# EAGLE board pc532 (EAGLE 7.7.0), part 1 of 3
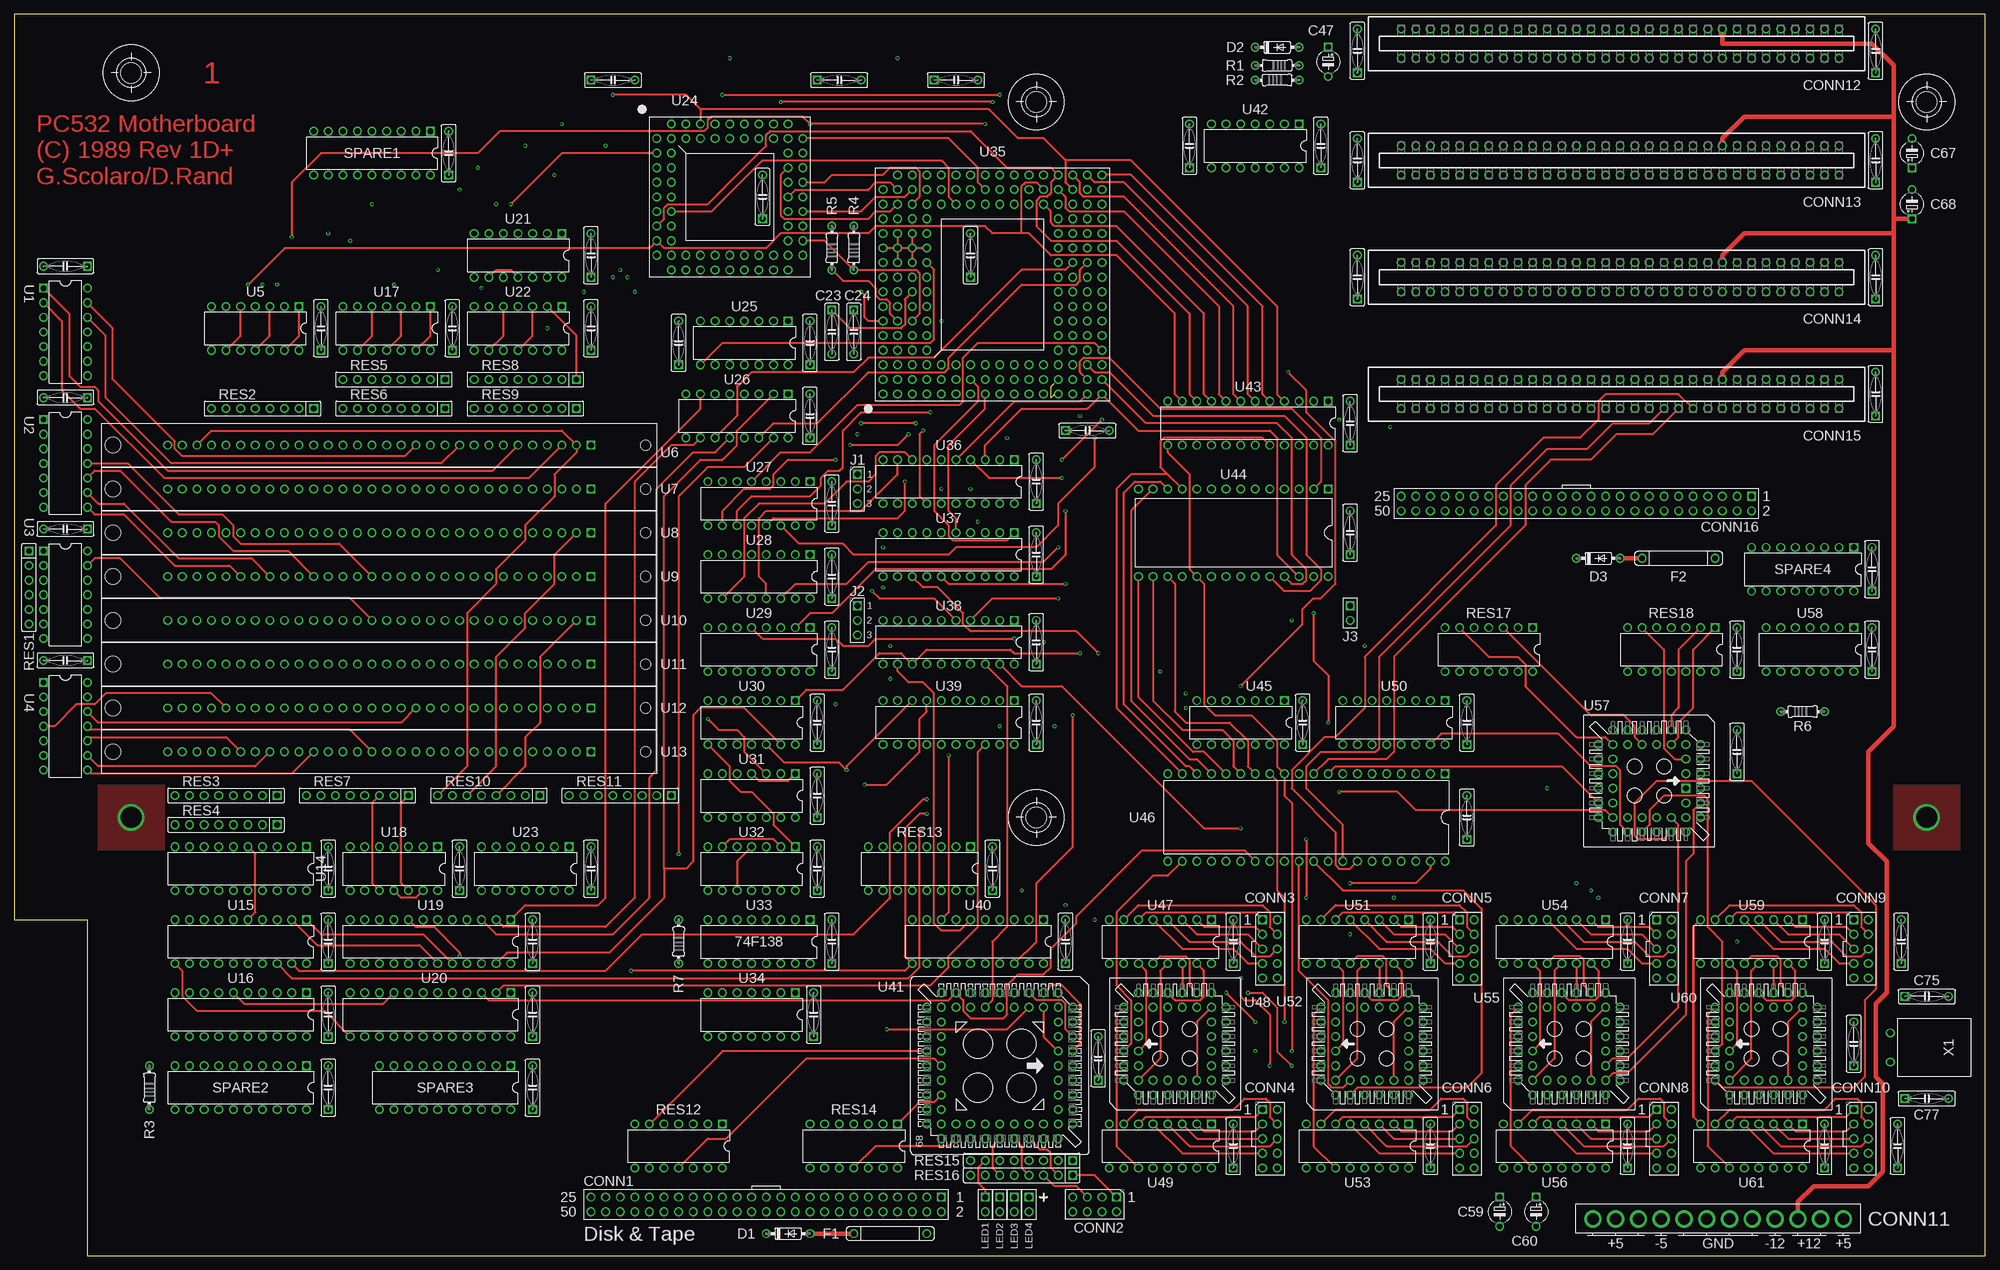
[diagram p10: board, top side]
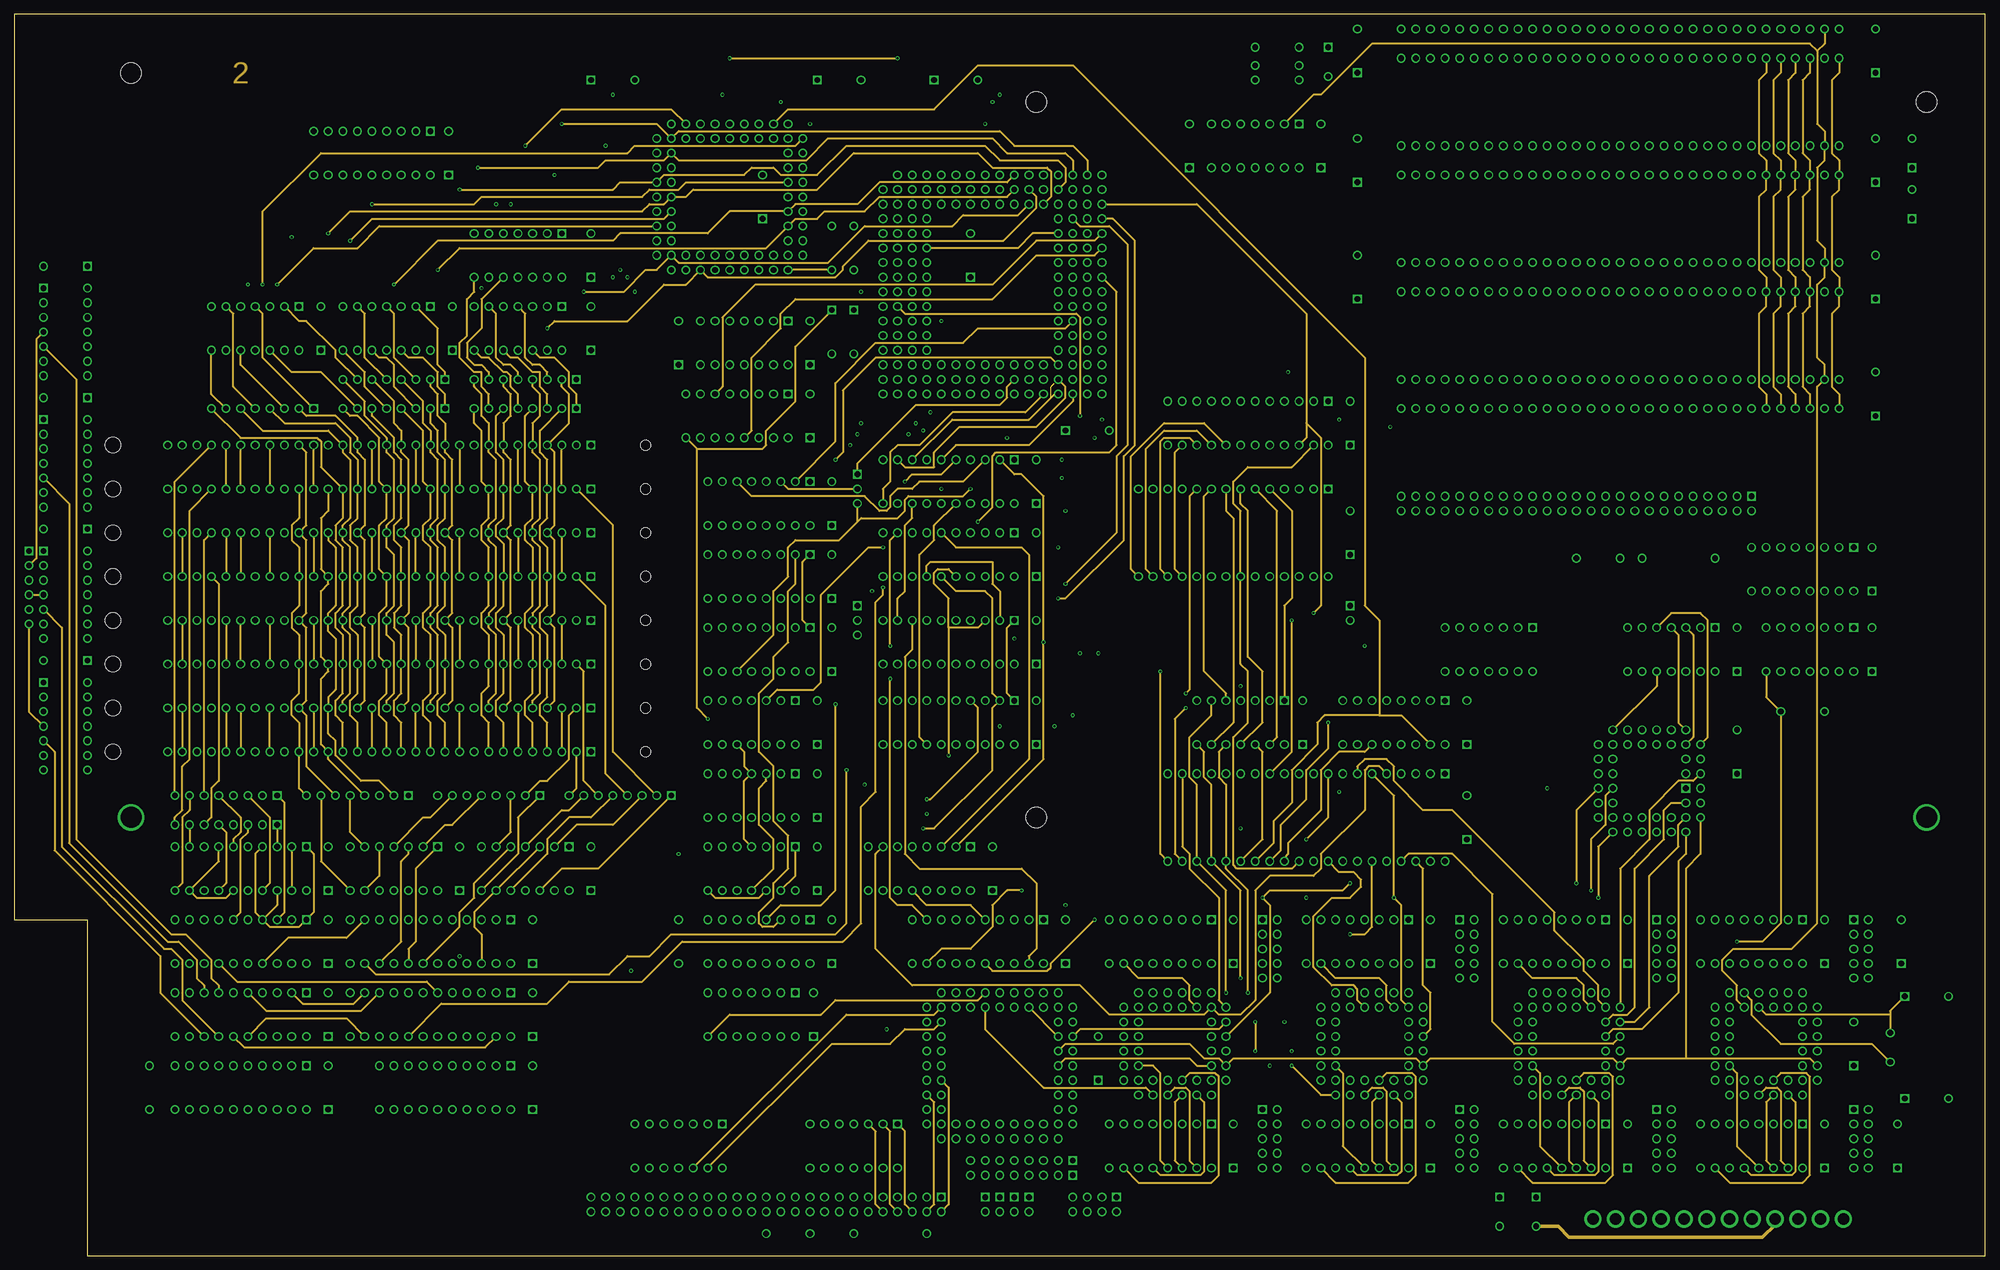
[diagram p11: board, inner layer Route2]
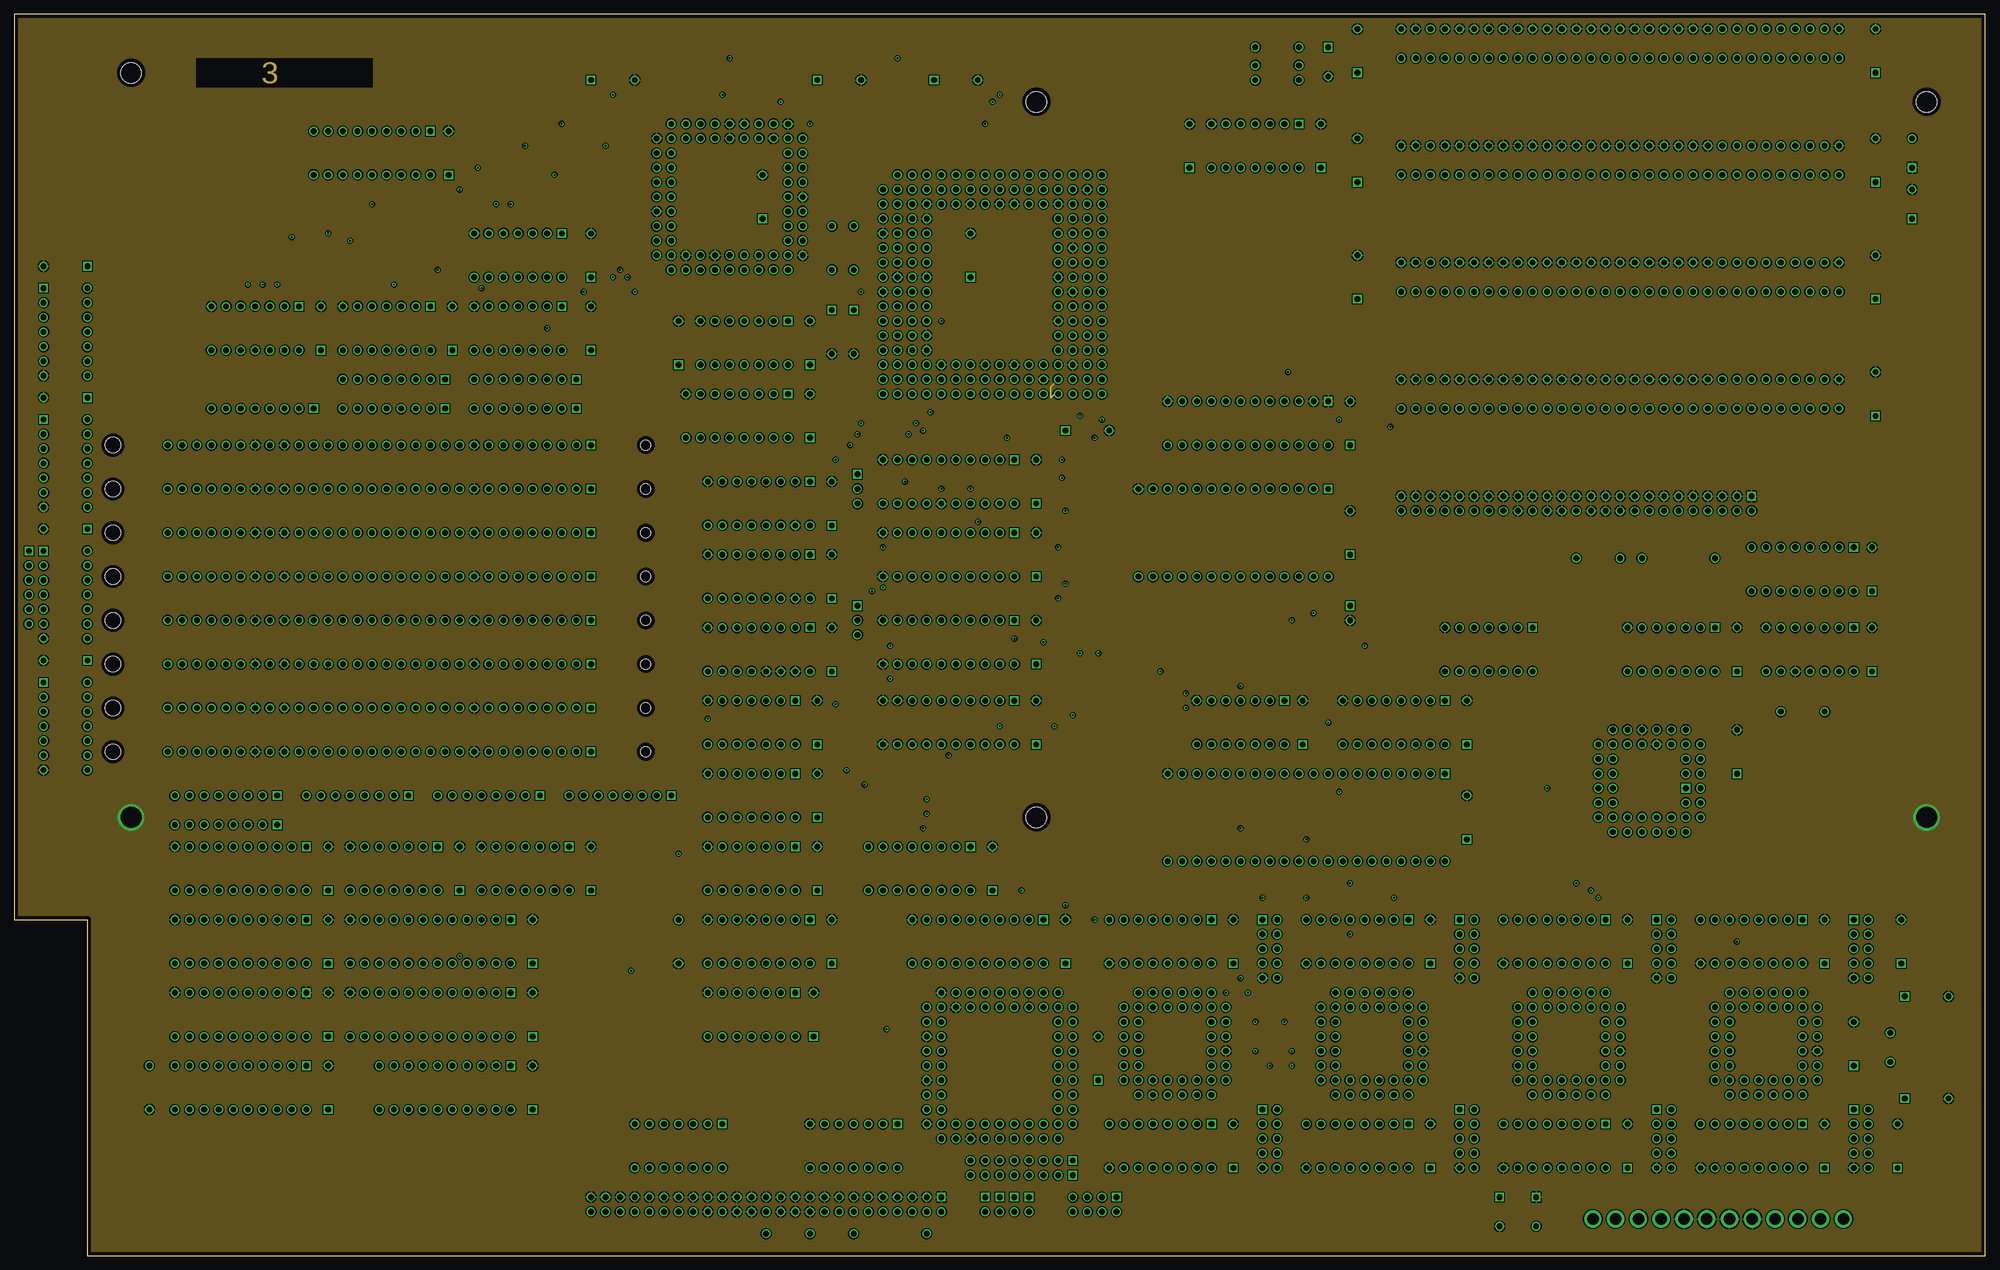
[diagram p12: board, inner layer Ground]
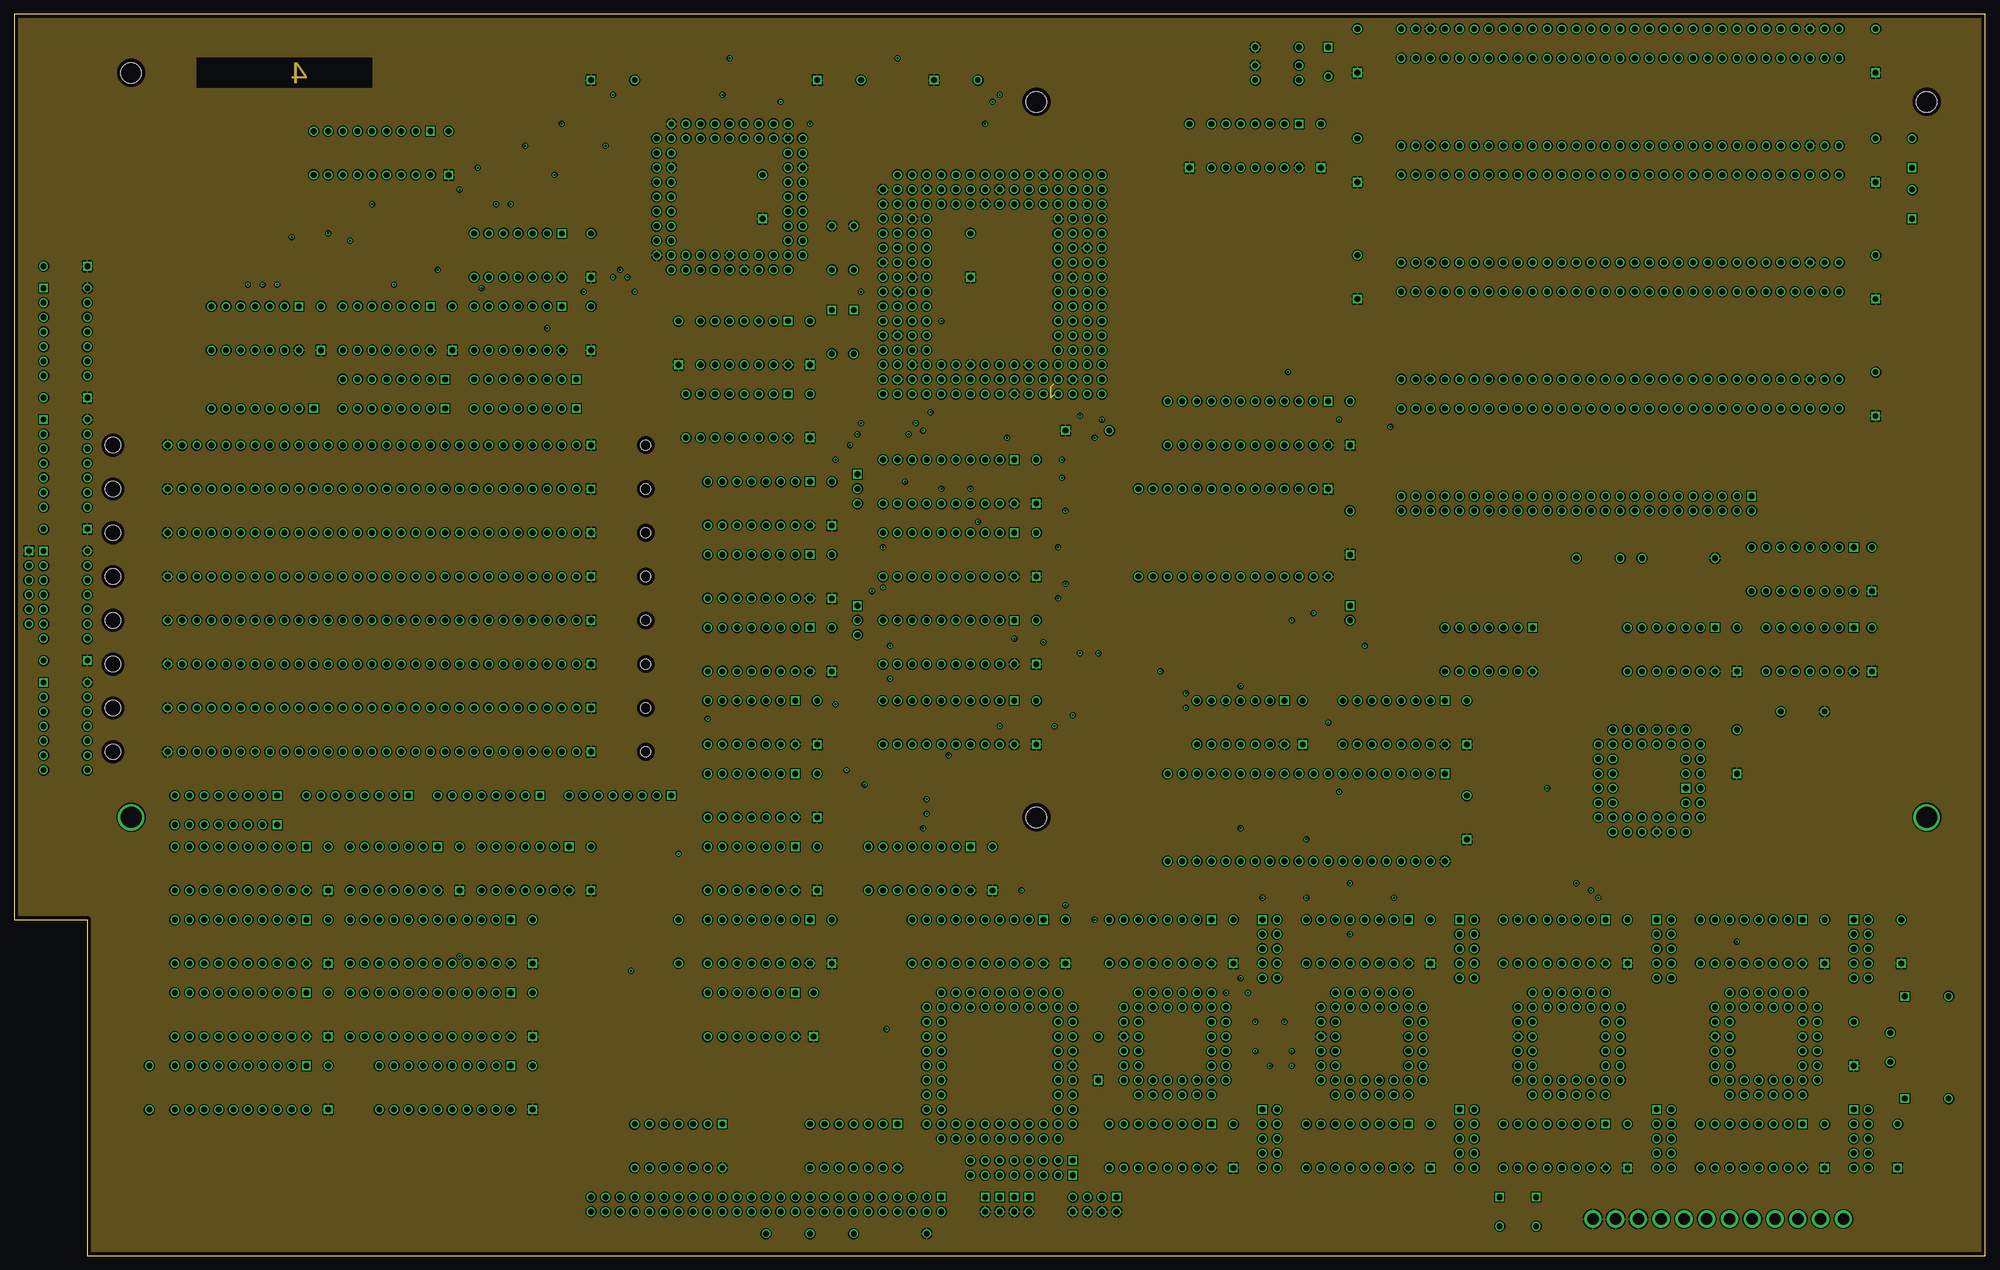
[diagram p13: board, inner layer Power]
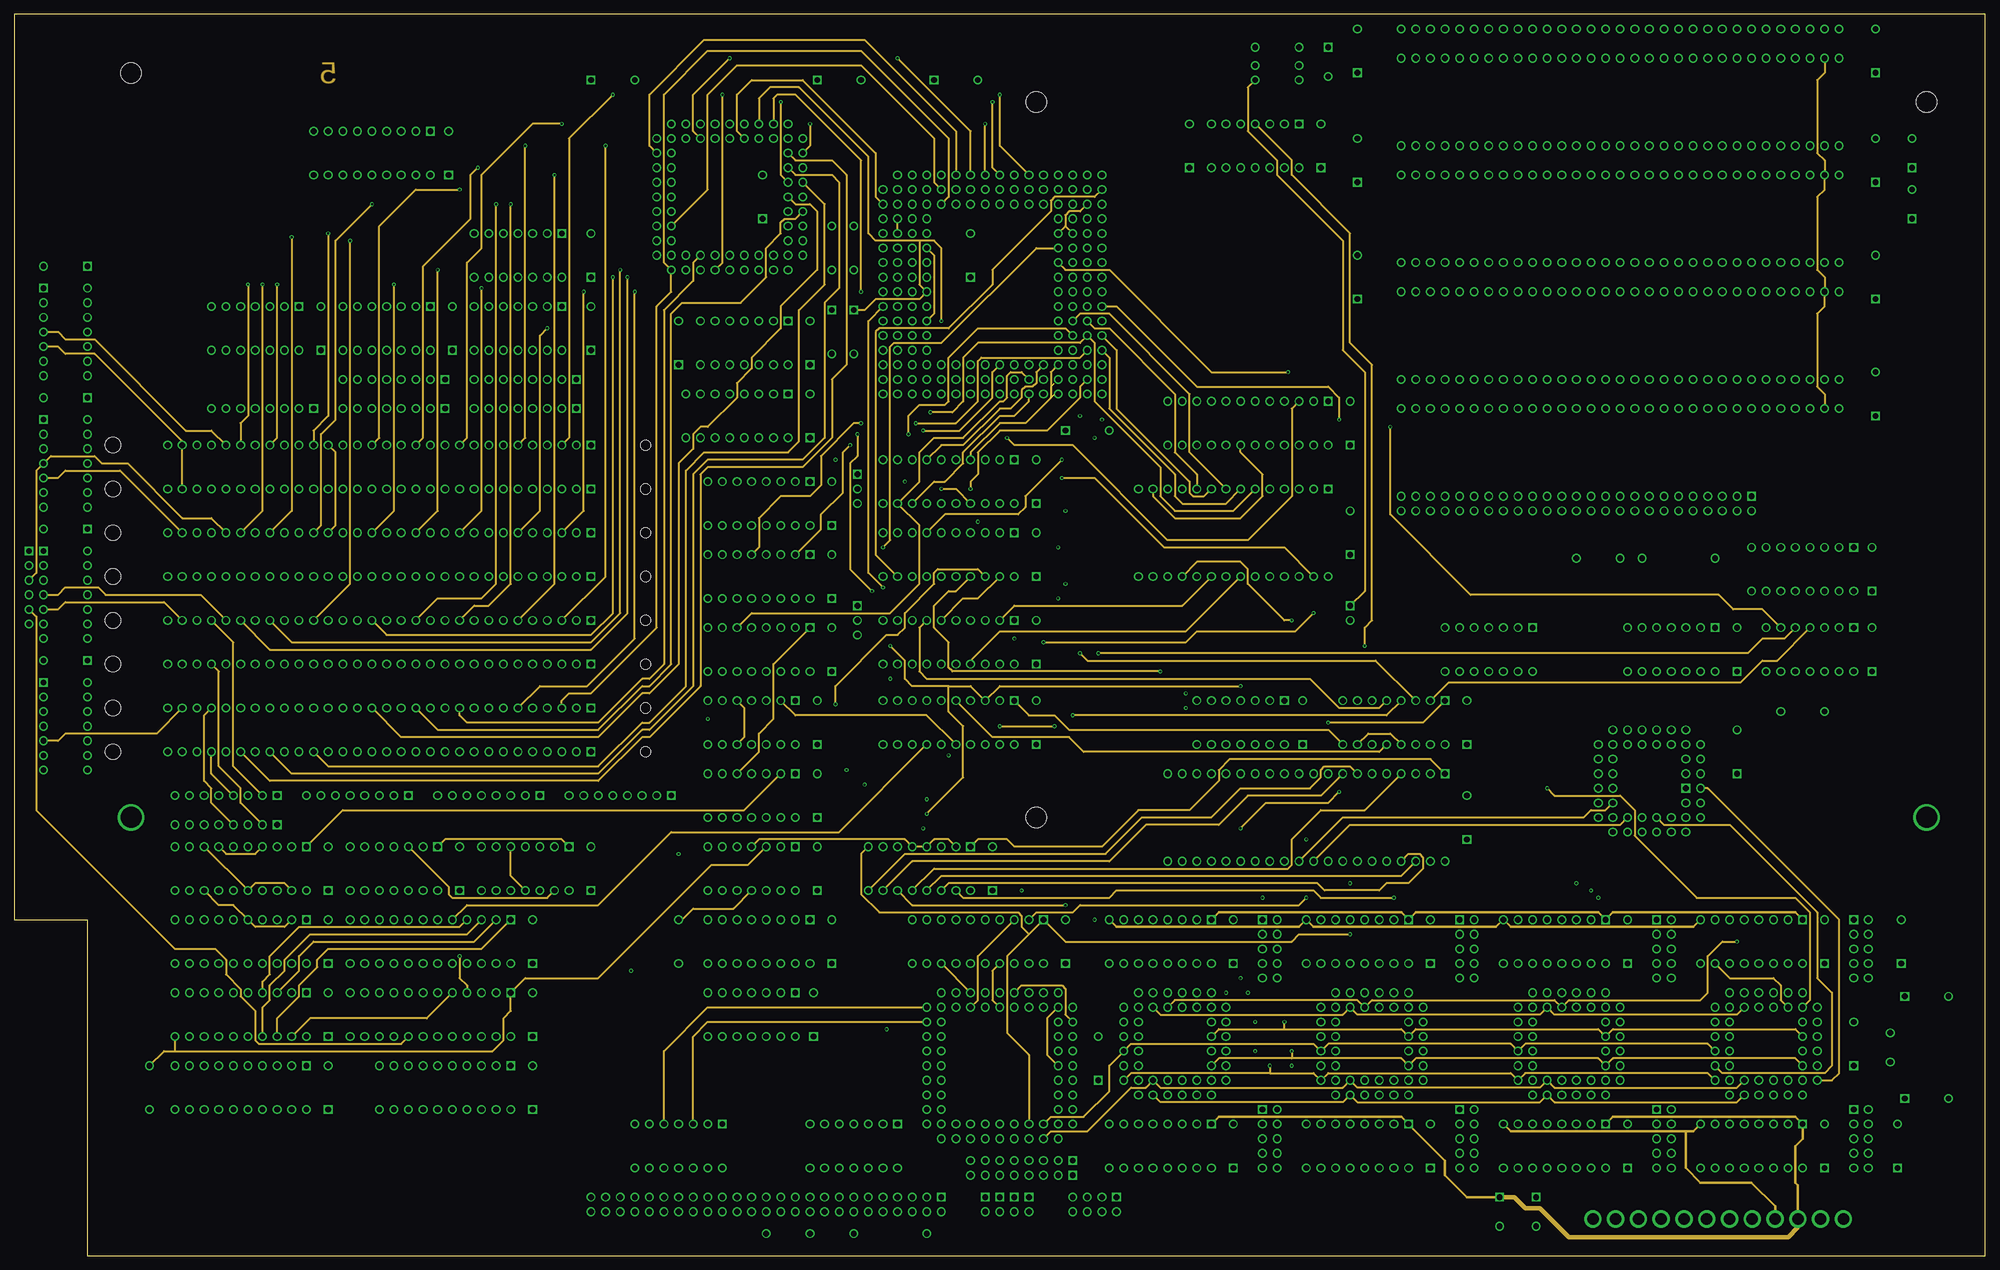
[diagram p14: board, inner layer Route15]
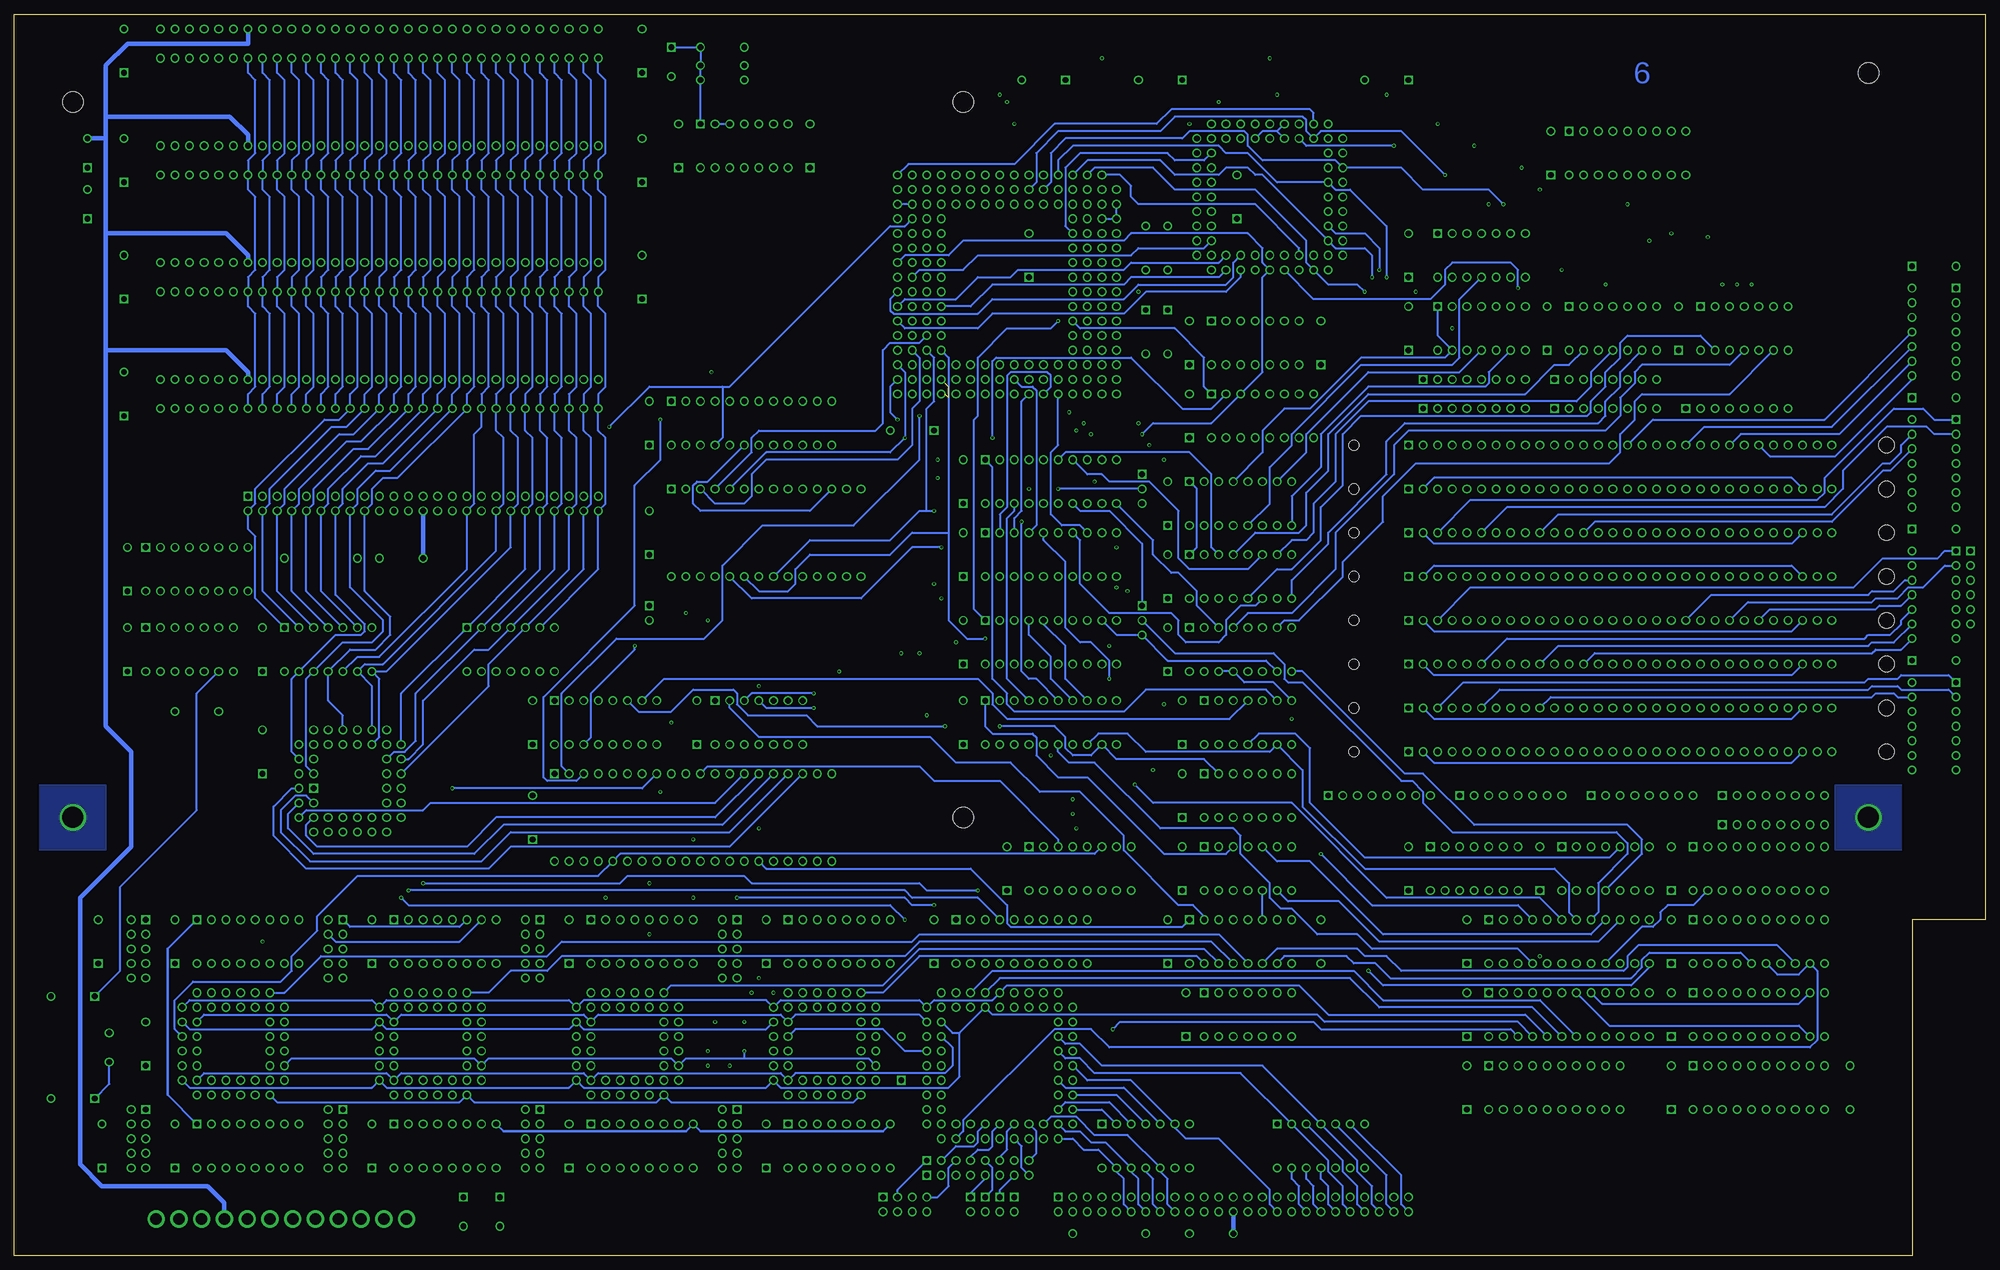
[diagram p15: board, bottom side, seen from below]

Size 342.9 x 215.9 mm. Coordinates in mm from the lower left corner, seen from the top.
Outline: 0,58.42 12.7,58.42 12.7,0 342.9,0 342.9,215.9 0,215.9 0,58.42
Copper layers (1*(2*3*14*15)*16): Top 0.035mm / dielectric 1.5mm / Route2 0.035mm / dielectric 0.15mm / Ground 0.035mm / dielectric 0.2mm / Power 0.035mm / dielectric 0.15mm / Route15 0.035mm / dielectric 0.2mm / Bottom 0.035mm
Design rules "ITEADstudio_DRC *": minimum track width 6mil, minimum drill 13mil, track to track 8mil, track to pad 8mil, pad to pad 8mil, via to via 8mil, smd to smd 0mil, copper to edge 25mil, drill to drill 10mil, minimum pad ring 10mil, minimum via ring 6mil, stop-mask expansion 2mil, vias tented up to drill 13mil, thermal gap 10mil
Net classes: 0 default: width 0.203 mm, drill 0.33 mm, clearance 0.203 mm; 1 power: width 0.813 mm, drill 0.33 mm, clearance 0.203 mm
Holes 3.6 mm at 20.32,205.74 332.74,200.66 177.8,200.66 177.8,76.2

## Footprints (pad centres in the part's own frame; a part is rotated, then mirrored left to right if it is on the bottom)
C_TH_300MIL = drill 1 square: 1 -3.81,0 | drill 1: 2 3.81,0
C_CYL_5X4MX = drill 1 square: + -2.54,0 | drill 1: - 2.54,0
HDR_2X25 = drill 1 square: 1 -30.48,-1.27 | drill 1: 2 -30.48,1.27; 3 -27.94,-1.27; 4 -27.94,1.27; 5 -25.4,-1.27; 6 -25.4,1.27; 7 -22.86,-1.27; 8 -22.86,1.27; 9 -20.32,-1.27; 10 -20.32,1.27; 11 -17.78,-1.27; 12 -17.78,1.27; 13 -15.24,-1.27; 14 -15.24,1.27; 15 -12.7,-1.27; 16 -12.7,1.27; 17 -10.16,-1.27; 18 -10.16,1.27; 19 -7.62,-1.27; 20 -7.62,1.27; 21 -5.08,-1.27; 22 -5.08,1.27; 23 -2.54,-1.27; 24 -2.54,1.27; 25 0,-1.27; 26 0,1.27; 27 2.54,-1.27; 28 2.54,1.27; 29 5.08,-1.27; 30 5.08,1.27; 31 7.62,-1.27; 32 7.62,1.27; 33 10.16,-1.27; 34 10.16,1.27; 35 12.7,-1.27; 36 12.7,1.27; 37 15.24,-1.27; 38 15.24,1.27; 39 17.78,-1.27; 40 17.78,1.27; 41 20.32,-1.27; 42 20.32,1.27; 43 22.86,-1.27; 44 22.86,1.27; 45 25.4,-1.27; 46 25.4,1.27; 47 27.94,-1.27; 48 27.94,1.27; 49 30.48,-1.27; 50 30.48,1.27
HDR_2X5 = drill 1 square: 1 -3.81,-1.27 | drill 1: 2 -3.81,1.27; 3 -1.27,-1.27; 4 -1.27,1.27; 5 1.27,-1.27; 6 1.27,1.27; 7 3.81,-1.27; 8 3.81,1.27
HDR_2X5' = drill 1 square: 1 -5.08,-1.27 | drill 1: 2 -5.08,1.27; 3 -2.54,-1.27; 4 -2.54,1.27; 5 0,-1.27; 6 0,1.27; 7 2.54,-1.27; 8 2.54,1.27; 9 5.08,-1.27; 10 5.08,1.27
AT_POWER = drill 2: P8-1 21.793,0; P8-2 17.831,0; P8-3 13.868,0; P8-4 9.906,0; P8-5 5.944,0; P8-6 1.981,0; P9-1 -1.981,0; P9-2 -5.944,0; P9-3 -9.906,0; P9-4 -13.868,0; P9-5 -17.831,0; P9-6 -21.793,0
ISA_SLOT8 = drill 1: A1 40.64,-2.54; A2 38.1,-2.54; A3 35.56,-2.54; A4 33.02,-2.54; A5 30.48,-2.54; A6 27.94,-2.54; A7 25.4,-2.54; A8 22.86,-2.54; A9 20.32,-2.54; A10 17.78,-2.54; A11 15.24,-2.54; A12 12.7,-2.54; A13 10.16,-2.54; A14 7.62,-2.54; A15 5.08,-2.54; A16 2.54,-2.54; A17 0,-2.54; A18 -2.54,-2.54; A19 -5.08,-2.54; A20 -7.62,-2.54; A21 -10.16,-2.54; A22 -12.7,-2.54; A23 -15.24,-2.54; A24 -17.78,-2.54; A25 -20.32,-2.54; A26 -22.86,-2.54; A27 -25.4,-2.54; A28 -27.94,-2.54; A29 -30.48,-2.54; A30 -33.02,-2.54; A31 -35.56,-2.54; B1 40.64,2.54; B2 38.1,2.54; B3 35.56,2.54; B4 33.02,2.54; B5 30.48,2.54; B6 27.94,2.54; B7 25.4,2.54; B8 22.86,2.54; B9 20.32,2.54; B10 17.78,2.54; B11 15.24,2.54; B12 12.7,2.54; B13 10.16,2.54; B14 7.62,2.54; B15 5.08,2.54; B16 2.54,2.54; B17 0,2.54; B18 -2.54,2.54; B19 -5.08,2.54; B20 -7.62,2.54; B21 -10.16,2.54; B22 -12.7,2.54; B23 -15.24,2.54; B24 -17.78,2.54; B25 -20.32,2.54; B26 -22.86,2.54; B27 -25.4,2.54; B28 -27.94,2.54; B29 -30.48,2.54; B30 -33.02,2.54; B31 -35.56,2.54
DO35 = drill 1: A 3.81,0; C -3.81,0
FUSE = drill 1: 1 -6.35,0; 2 6.35,0
HDR_1X3 = drill 1 square: 1 -2.54,0 | drill 1: 2 0,0; 3 2.54,0
HDR_1X2 = drill 1 square: 1 -1.27,0 | drill 1: 2 1.27,0
LED_JUMPER = drill 1 square: 1 -1.27,0 | drill 1: 2 1.27,0
R_204/7 = drill 1: 1 -3.81,0; 2 3.81,0
RN_SIP6 = drill 1 pad 1.4 square: 1 -6.35,0 | drill 1 pad 1.4: 2 -3.81,0; 3 -1.27,0; 4 1.27,0; 5 3.81,0; 6 6.35,0
RN_SIP8 = drill 1 square: 1 0,0 | drill 1: 2 -2.54,0; 3 -5.08,0; 4 -7.62,0; 5 -10.16,0; 6 -12.7,0; 7 -15.24,0; 8 -17.78,0
DIL14 = drill 1 square: 1 -7.62,-3.81 | drill 1: 2 -5.08,-3.81; 3 -2.54,-3.81; 4 0,-3.81; 5 2.54,-3.81; 6 5.08,-3.81; 7 7.62,-3.81; 8 7.62,3.81; 9 5.08,3.81; 10 2.54,3.81; 11 0,3.81; 12 -2.54,3.81; 13 -5.08,3.81; 14 -7.62,3.81
DIL16 = drill 1 square: 1 -8.89,-3.81 | drill 1: 2 -6.35,-3.81; 3 -3.81,-3.81; 4 -1.27,-3.81; 5 1.27,-3.81; 6 3.81,-3.81; 7 6.35,-3.81; 8 8.89,-3.81; 9 8.89,3.81; 10 6.35,3.81; 11 3.81,3.81; 12 1.27,3.81; 13 -1.27,3.81; 14 -3.81,3.81; 15 -6.35,3.81; 16 -8.89,3.81
DIL18 = drill 1 square: 1 -10.16,-3.81 | drill 1: 2 -7.62,-3.81; 3 -5.08,-3.81; 4 -2.54,-3.81; 5 0,-3.81; 6 2.54,-3.81; 7 5.08,-3.81; 8 7.62,-3.81; 9 10.16,-3.81; 10 10.16,3.81; 11 7.62,3.81; 12 5.08,3.81; 13 2.54,3.81; 14 0,3.81; 15 -2.54,3.81; 16 -5.08,3.81; 17 -7.62,3.81; 18 -10.16,3.81
DIL20 = drill 1 square: 1 -11.43,-3.81 | drill 1: 2 -8.89,-3.81; 3 -6.35,-3.81; 4 -3.81,-3.81; 5 -1.27,-3.81; 6 1.27,-3.81; 7 3.81,-3.81; 8 6.35,-3.81; 9 8.89,-3.81; 10 11.43,-3.81; 11 11.43,3.81; 12 8.89,3.81; 13 6.35,3.81; 14 3.81,3.81; 15 1.27,3.81; 16 -1.27,3.81; 17 -3.81,3.81; 18 -6.35,3.81; 19 -8.89,3.81; 20 -11.43,3.81
SIMM_30 = drill 1 square: 1 36.83,0 | drill 1: 2 34.29,0; 3 31.75,0; 4 29.21,0; 5 26.67,0; 6 24.13,0; 7 21.59,0; 8 19.05,0; 9 16.51,0; 10 13.97,0; 11 11.43,0; 12 8.89,0; 13 6.35,0; 14 3.81,0; 15 1.27,0; 16 -1.27,0; 17 -3.81,0; 18 -6.35,0; 19 -8.89,0; 20 -11.43,0; 21 -13.97,0; 22 -16.51,0; 23 -19.05,0; 24 -21.59,0; 25 -24.13,0; 26 -26.67,0; 27 -29.21,0; 28 -31.75,0; 29 -34.29,0; 30 -36.83,0 | hole 2.7: -46.355,0 | hole 1.8: 46.355,0
DIL20_ROUND = drill 1 square: 1 -11.43,-3.81 | drill 1: 2 -8.89,-3.81; 3 -6.35,-3.81; 4 -3.81,-3.81; 5 -1.27,-3.81; 6 1.27,-3.81; 7 3.81,-3.81; 8 6.35,-3.81; 9 8.89,-3.81; 10 11.43,-3.81; 11 11.43,3.81; 12 8.89,3.81; 13 6.35,3.81; 14 3.81,3.81; 15 1.27,3.81; 16 -1.27,3.81; 17 -3.81,3.81; 18 -6.35,3.81; 19 -8.89,3.81; 20 -11.43,3.81
DIL24 = drill 1 square: 1 -13.97,-3.81 | drill 1: 2 -11.43,-3.81; 3 -8.89,-3.81; 4 -6.35,-3.81; 5 -3.81,-3.81; 6 -1.27,-3.81; 7 1.27,-3.81; 8 3.81,-3.81; 9 6.35,-3.81; 10 8.89,-3.81; 11 11.43,-3.81; 12 13.97,-3.81; 13 13.97,3.81; 14 11.43,3.81; 15 8.89,3.81; 16 6.35,3.81; 17 3.81,3.81; 18 1.27,3.81; 19 -1.27,3.81; 20 -3.81,3.81; 21 -6.35,3.81; 22 -8.89,3.81; 23 -11.43,3.81; 24 -13.97,3.81
PGA68 = drill 1: A2 -10.16,12.7; A3 -7.62,12.7; A4 -5.08,12.7; A5 -2.54,12.7; A6 0,12.7; A7 2.54,12.7; A8 5.08,12.7; A9 7.62,12.7; A10 10.16,12.7; B1 -12.7,10.16; B2 -10.16,10.16; B3 -7.62,10.16; B4 -5.08,10.16; B5 -2.54,10.16; B6 0,10.16; B7 2.54,10.16; B8 5.08,10.16; B9 7.62,10.16; B10 10.16,10.16; B11 12.7,10.16; C1 -12.7,7.62; C2 -10.16,7.62; C10 10.16,7.62; C11 12.7,7.62; D1 -12.7,5.08; D2 -10.16,5.08; D10 10.16,5.08; D11 12.7,5.08; E1 -12.7,2.54; E2 -10.16,2.54; E10 10.16,2.54; E11 12.7,2.54; F1 -12.7,0; F2 -10.16,0; F10 10.16,0; F11 12.7,0; G1 -12.7,-2.54; G2 -10.16,-2.54; G10 10.16,-2.54; G11 12.7,-2.54; H1 -12.7,-5.08; H2 -10.16,-5.08; H10 10.16,-5.08; H11 12.7,-5.08; J1 -12.7,-7.62; J2 -10.16,-7.62; J10 10.16,-7.62; J11 12.7,-7.62; K1 -12.7,-10.16; K2 -10.16,-10.16; K3 -7.62,-10.16; K4 -5.08,-10.16; K5 -2.54,-10.16; K6 0,-10.16; K7 2.54,-10.16; K8 5.08,-10.16; K9 7.62,-10.16; K10 10.16,-10.16; K11 12.7,-10.16; L2 -10.16,-12.7; L3 -7.62,-12.7; L4 -5.08,-12.7; L5 -2.54,-12.7; L6 0,-12.7; L7 2.54,-12.7; L8 5.08,-12.7; L9 7.62,-12.7; L10 10.16,-12.7
PGA175 = drill 1: A1 -19.05,19.05; A2 -16.51,19.05; A3 -13.97,19.05; A4 -11.43,19.05; A5 -8.89,19.05; A6 -6.35,19.05; A7 -3.81,19.05; A8 -1.27,19.05; A9 1.27,19.05; A10 3.81,19.05; A11 6.35,19.05; A12 8.89,19.05; A13 11.43,19.05; A14 13.97,19.05; A15 16.51,19.05; B1 -19.05,16.51; B2 -16.51,16.51; B3 -13.97,16.51; B4 -11.43,16.51; B5 -8.89,16.51; B6 -6.35,16.51; B7 -3.81,16.51; B8 -1.27,16.51; B9 1.27,16.51; B10 3.81,16.51; B11 6.35,16.51; B12 8.89,16.51; B13 11.43,16.51; B14 13.97,16.51; B15 16.51,16.51; B16 19.05,16.51; C1 -19.05,13.97; C2 -16.51,13.97; C3 -13.97,13.97; C4 -11.43,13.97; C5 -8.89,13.97; C6 -6.35,13.97; C7 -3.81,13.97; C8 -1.27,13.97; C9 1.27,13.97; C10 3.81,13.97; C11 6.35,13.97; C12 8.89,13.97; C13 11.43,13.97; C14 13.97,13.97; C15 16.51,13.97; C16 19.05,13.97; D1 -19.05,11.43; D2 -16.51,11.43; D3 -13.97,11.43; D4 -11.43,11.43; D5 -8.89,11.43; D6 -6.35,11.43; D7 -3.81,11.43; D8 -1.27,11.43; D9 1.27,11.43; D10 3.81,11.43; D11 6.35,11.43; D12 8.89,11.43; D13 11.43,11.43; D14 13.97,11.43; D15 16.51,11.43; D16 19.05,11.43; E1 -19.05,8.89; E2 -16.51,8.89; E3 -13.97,8.89; E14 13.97,8.89; E15 16.51,8.89; E16 19.05,8.89; F1 -19.05,6.35; F2 -16.51,6.35; F3 -13.97,6.35; F14 13.97,6.35; F15 16.51,6.35; F16 19.05,6.35; G1 -19.05,3.81; G2 -16.51,3.81; G3 -13.97,3.81; G14 13.97,3.81; G15 16.51,3.81; G16 19.05,3.81; H1 -19.05,1.27; H2 -16.51,1.27; H3 -13.97,1.27; H14 13.97,1.27; H15 16.51,1.27; H16 19.05,1.27; J1 -19.05,-1.27; J2 -16.51,-1.27; J3 -13.97,-1.27; J14 13.97,-1.27; J15 16.51,-1.27; J16 19.05,-1.27; K1 -19.05,-3.81; K2 -16.51,-3.81; K3 -13.97,-3.81; K14 13.97,-3.81; K15 16.51,-3.81; K16 19.05,-3.81; L1 -19.05,-6.35; L2 -16.51,-6.35; L3 -13.97,-6.35; L14 13.97,-6.35; L15 16.51,-6.35; L16 19.05,-6.35; M1 -19.05,-8.89; M2 -16.51,-8.89; M3 -13.97,-8.89; M14 13.97,-8.89; M15 16.51,-8.89; M16 19.05,-8.89; N1 -16.51,-11.43; N2 -19.05,-11.43; N3 -13.97,-11.43; N4 -11.43,-11.43; N5 -8.89,-11.43; N6 -6.35,-11.43; N7 -3.81,-11.43; N8 -1.27,-11.43; N9 1.27,-11.43; N10 3.81,-11.43; N11 6.35,-11.43; N12 8.89,-11.43; N13 11.43,-11.43; N14 13.97,-11.43; N15 16.51,-11.43; N16 19.05,-11.43; P1 -19.05,-13.97; P2 -16.51,-13.97; P3 -13.97,-13.97; P4 -11.43,-13.97; P5 -8.89,-13.97; P6 -6.35,-13.97; P7 -3.81,-13.97; P8 -1.27,-13.97; P9 1.27,-13.97; P10 3.81,-13.97; P11 6.35,-13.97; P12 8.89,-13.97; P13 11.43,-13.97; P14 13.97,-13.97; P15 16.51,-13.97; P16 19.05,-13.97; R1 -19.05,-16.51; R2 -16.51,-16.51; R3 -13.97,-16.51; R4 -11.43,-16.51; R5 -8.89,-16.51; R6 -6.35,-16.51; R7 -3.81,-16.51; R8 -1.27,-16.51; R9 1.27,-16.51; R10 3.81,-16.51; R11 6.35,-16.51; R12 8.89,-16.51; R13 11.43,-16.51; R14 13.97,-16.51; R15 16.51,-16.51; R16 19.05,-16.51; S1 -19.05,-19.05; S2 -16.51,-19.05; S3 -13.97,-19.05; S4 -11.43,-19.05; S5 -8.89,-19.05; S6 -6.35,-19.05; S7 -3.81,-19.05; S8 -1.27,-19.05; S9 1.27,-19.05; S10 3.81,-19.05; S11 6.35,-19.05; S12 8.89,-19.05; S13 11.43,-19.05; S14 13.97,-19.05; S15 16.51,-19.05; S16 19.05,-19.05
PLCC68 = drill 1: 1 0,12.7; 2 0,10.16; 3 -2.54,12.7; 4 -2.54,10.16; 5 -5.08,12.7; 6 -5.08,10.16; 7 -7.62,12.7; 8 -7.62,10.16; 9 -10.16,12.7; 10 -12.7,10.16; 11 -10.16,10.16; 12 -12.7,7.62; 13 -10.16,7.62; 14 -12.7,5.08; 15 -10.16,5.08; 16 -12.7,2.54; 17 -10.16,2.54; 18 -12.7,0; 19 -10.16,0; 20 -12.7,-2.54; 21 -10.16,-2.54; 22 -12.7,-5.08; 23 -10.16,-5.08; 24 -12.7,-7.62; 25 -10.16,-7.62; 26 -12.7,-10.16; 27 -10.16,-12.7; 28 -10.16,-10.16; 29 -7.62,-12.7; 30 -7.62,-10.16; 31 -5.08,-12.7; 32 -5.08,-10.16; 33 -2.54,-12.7; 34 -2.54,-10.16; 35 0,-12.7; 36 0,-10.16; 37 2.54,-12.7; 38 2.54,-10.16; 39 5.08,-12.7; 40 5.08,-10.16; 41 7.62,-12.7; 42 7.62,-10.16; 43 10.16,-12.7; 44 12.7,-10.16; 45 10.16,-10.16; 46 12.7,-7.62; 47 10.16,-7.62; 48 12.7,-5.08; 49 10.16,-5.08; 50 12.7,-2.54; 51 10.16,-2.54; 52 12.7,0; 53 10.16,0; 54 12.7,2.54; 55 10.16,2.54; 56 12.7,5.08; 57 10.16,5.08; 58 12.7,7.62; 59 10.16,7.62; 60 12.7,10.16; 61 10.16,12.7; 62 10.16,10.16; 63 7.62,12.7; 64 7.62,10.16; 65 5.08,12.7; 66 5.08,10.16; 67 2.54,12.7; 68 2.54,10.16
DIL28W = drill 1 pad 1.4 square: 1 -16.51,-7.62 | drill 1 pad 1.4: 2 -13.97,-7.62; 3 -11.43,-7.62; 4 -8.89,-7.62; 5 -6.35,-7.62; 6 -3.81,-7.62; 7 -1.27,-7.62; 8 1.27,-7.62; 9 3.81,-7.62; 10 6.35,-7.62; 11 8.89,-7.62; 12 11.43,-7.62; 13 13.97,-7.62; 14 16.51,-7.62; 15 16.51,7.62; 16 13.97,7.62; 17 11.43,7.62; 18 8.89,7.62; 19 6.35,7.62; 20 3.81,7.62; 21 1.27,7.62; 22 -1.27,7.62; 23 -3.81,7.62; 24 -6.35,7.62; 25 -8.89,7.62; 26 -11.43,7.62; 27 -13.97,7.62; 28 -16.51,7.62
DIL40 = drill 1 square: 1 -22.86,-7.62 | drill 1: 2 -20.32,-7.62; 3 -17.78,-7.62; 4 -15.24,-7.62; 5 -12.7,-7.62; 6 -10.16,-7.62; 7 -7.62,-7.62; 8 -5.08,-7.62; 9 -2.54,-7.62; 10 0,-7.62; 11 2.54,-7.62; 12 5.08,-7.62; 13 7.62,-7.62; 14 10.16,-7.62; 15 12.7,-7.62; 16 15.24,-7.62; 17 17.78,-7.62; 18 20.32,-7.62; 19 22.86,-7.62; 20 25.4,-7.62; 21 25.4,7.62; 22 22.86,7.62; 23 20.32,7.62; 24 17.78,7.62; 25 15.24,7.62; 26 12.7,7.62; 27 10.16,7.62; 28 7.62,7.62; 29 5.08,7.62; 30 2.54,7.62; 31 0,7.62; 32 -2.54,7.62; 33 -5.08,7.62; 34 -7.62,7.62; 35 -10.16,7.62; 36 -12.7,7.62; 37 -15.24,7.62; 38 -17.78,7.62; 39 -20.32,7.62; 40 -22.86,7.62
PLCC44 = drill 1: 1 1.27,6.35; 2 -1.27,8.89; 3 -1.27,6.35; 4 -3.81,8.89; 5 -3.81,6.35; 6 -6.35,8.89; 7 -8.89,6.35; 8 -6.35,6.35; 9 -8.89,3.81; 10 -6.35,3.81; 11 -8.89,1.27; 12 -6.35,1.27; 13 -8.89,-1.27; 14 -6.35,-1.27; 15 -8.89,-3.81; 16 -6.35,-3.81; 17 -8.89,-6.35; 18 -6.35,-8.89; 19 -6.35,-6.35; 20 -3.81,-8.89; 21 -3.81,-6.35; 22 -1.27,-8.89; 23 -1.27,-6.35; 24 1.27,-8.89; 25 1.27,-6.35; 26 3.81,-8.89; 27 3.81,-6.35; 28 6.35,-8.89; 29 8.89,-6.35; 30 6.35,-6.35; 31 8.89,-3.81; 32 6.35,-3.81; 33 8.89,-1.27; 34 6.35,-1.27; 35 8.89,1.27; 36 6.35,1.27; 37 8.89,3.81; 38 6.35,3.81; 39 8.89,6.35; 40 6.35,8.89; 41 6.35,6.35; 42 3.81,8.89; 43 3.81,6.35; 44 1.27,8.89
PLCC44' = drill 1 square: 1 1.27,6.35 | drill 1: 2 -1.27,8.89; 3 -1.27,6.35; 4 -3.81,8.89; 5 -3.81,6.35; 6 -6.35,8.89; 7 -8.89,6.35; 8 -6.35,6.35; 9 -8.89,3.81; 10 -6.35,3.81; 11 -8.89,1.27; 12 -6.35,1.27; 13 -8.89,-1.27; 14 -6.35,-1.27; 15 -8.89,-3.81; 16 -6.35,-3.81; 17 -8.89,-6.35; 18 -6.35,-8.89; 19 -6.35,-6.35; 20 -3.81,-8.89; 21 -3.81,-6.35; 22 -1.27,-8.89; 23 -1.27,-6.35; 24 1.27,-8.89; 25 1.27,-6.35; 26 3.81,-8.89; 27 3.81,-6.35; 28 6.35,-8.89; 29 8.89,-6.35; 30 6.35,-6.35; 31 8.89,-3.81; 32 6.35,-3.81; 33 8.89,-1.27; 34 6.35,-1.27; 35 8.89,1.27; 36 6.35,1.27; 37 8.89,3.81; 38 6.35,3.81; 39 8.89,6.35; 40 6.35,8.89; 41 6.35,6.35; 42 3.81,8.89; 43 3.81,6.35; 44 1.27,8.89
XTAL = drill 1: 1 -2.54,-6.985; 2 2.54,-6.985

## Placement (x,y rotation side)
C1  .1uF  [C_TH_300MIL]  54.61,41.91 90 top
C2  .1uF  [C_TH_300MIL]  54.61,29.21 90 top
C3  .1uF  [C_TH_300MIL]  90.17,29.21 90 top
C4  .1uF  [C_TH_300MIL]  90.17,41.91 90 top
C5  .1uF  [C_TH_300MIL]  54.61,54.61 90 top
C6  .1uF  [C_TH_300MIL]  90.17,54.61 90 top
C7  .1uF  [C_TH_300MIL]  54.61,67.31 90 top
C8  .1uF  [C_TH_300MIL]  77.47,67.31 90 top
C9  .1uF  [C_TH_300MIL]  100.33,67.31 90 top
C10  .1uF  [C_TH_300MIL]  212.09,54.61 90 top
C11  .1uF  [C_TH_300MIL]  188.59,34.29 90 top
C12  .1uF  [C_TH_300MIL]  246.38,54.61 90 top
C13  .1uF  [C_TH_300MIL]  212.09,19.05 90 top
C14  .1uF  [C_TH_300MIL]  280.67,54.61 90 top
C15  .1uF  [C_TH_300MIL]  246.38,19.05 90 top
C16  .1uF  [C_TH_300MIL]  314.96,54.61 90 top
C17  .1uF  [C_TH_300MIL]  280.67,19.05 90 top
C18  .1uF  [C_TH_300MIL]  314.96,19.05 90 top
C19  .1uF  [C_TH_300MIL]  320.04,36.83 90 top
C20  .1uF  [C_TH_300MIL]  328.3,54.61 90 top
C21  .1uF  [C_TH_300MIL]  327.66,19.05 90 top
C22  .1uF  [C_TH_300MIL]  170.18,67.31 90 top
C23  50pF  [C_TH_300MIL]  142.24,160.66 270 top
C24  50pF  [C_TH_300MIL]  146.05,160.66 270 top
C25  .1uF  [C_TH_300MIL]  8.89,126.36 180 top
C26  .1uF  [C_TH_300MIL]  299.72,87.63 90 top
C27  .1uF  [C_TH_300MIL]  8.89,149.22 180 top
C28  .1uF  [C_TH_300MIL]  252.73,76.2 90 top
C29  .1uF  [C_TH_300MIL]  8.89,172.09 180 top
C30  .1uF  [C_TH_300MIL]  299.72,105.41 90 top
C31  .1uF  [C_TH_300MIL]  323.21,105.41 90 top
C32  .1uF  [C_TH_300MIL]  323.21,119.38 90 top
C33  .1uF  [C_TH_300MIL]  323.85,209.55 90 top
C34  .1uF  [C_TH_300MIL]  323.85,190.5 90 top
C35  .1uF  [C_TH_300MIL]  323.85,170.18 90 top
C36  .1uF  [C_TH_300MIL]  323.85,149.86 90 top
C37  .1uF  [C_TH_300MIL]  233.68,209.55 90 top
C38  .1uF  [C_TH_300MIL]  204.47,193.04 90 top
C39  .1uF  [C_TH_300MIL]  233.68,170.18 90 top
C40  .1uF  [C_TH_300MIL]  233.68,190.5 90 top
C41  .1uF  [C_TH_300MIL]  232.41,144.78 90 top
C42  .1uF  [C_TH_300MIL]  186.69,143.51 0 top
C43  .1uF  [C_TH_300MIL]  232.41,125.73 90 top
C44  .1uF  [C_TH_300MIL]  177.8,134.62 90 top
C45  .1uF  [C_TH_300MIL]  75.56,191.77 90 top
C46  .1uF  [C_TH_300MIL]  177.8,106.68 90 top
C47  33uF  [C_CYL_5X4MX]  228.6,207.65 270 top
C48  .1uF  [C_TH_300MIL]  177.8,92.71 90 top
C49  .1uF  [C_TH_300MIL]  227.33,193.04 90 top
C50  .1uF  [C_TH_300MIL]  104.14,204.47 0 top
C51  .1uF  [C_TH_300MIL]  53.34,161.29 90 top
C52  .1uF  [C_TH_300MIL]  100.33,173.99 90 top
C53  .1uF  [C_TH_300MIL]  76.2,161.29 90 top
C54  .1uF  [C_TH_300MIL]  100.33,161.29 90 top
C55  .1uF  [C_TH_300MIL]  142.24,54.61 90 top
C56  .1uF  [C_TH_300MIL]  139.06,41.91 90 top
C57  .1uF  [C_TH_300MIL]  139.7,67.31 90 top
C58  .1uF  [C_TH_300MIL]  139.7,92.71 90 top
C59  10uF  [C_CYL_5X4MX]  258.44,7.62 270 top
C60  10uF  [C_CYL_5X4MX]  264.8,7.62 270 top
C61  .1uF  [C_TH_300MIL]  142.24,130.81 90 top
C62  .1uF  [C_TH_300MIL]  142.24,105.41 90 top
C63  .1uF  [C_TH_300MIL]  115.57,158.75 90 top
C64  .1uF  [C_TH_300MIL]  138.43,146.05 90 top
C65  .1uF  [C_TH_300MIL]  138.43,158.75 90 top
C66  .1uF  [C_TH_300MIL]  166.37,173.99 90 top
C67  10uF  [C_CYL_5X4MX]  330.2,191.77 90 top
C68  10uF  [C_CYL_5X4MX]  330.2,182.88 90 top
C69  .1uF  [C_TH_300MIL]  130.18,184.15 90 top
C70  .1uF  [C_TH_300MIL]  252.73,92.71 90 top
C71  .1uF  [C_TH_300MIL]  224.16,92.71 90 top
C72  .1uF  [C_TH_300MIL]  177.8,121.92 90 top
C73  .1uF  [C_TH_300MIL]  8.89,103.5 180 top
C74  .1uF  [C_TH_300MIL]  182.88,54.61 90 top
C75  10pF  [C_TH_300MIL]  332.74,45.09 0 top
C76  .1uF  [C_TH_300MIL]  142.24,118.11 90 top
C77  5pF  [C_TH_300MIL]  332.74,27.3 0 top
C78  .1uF  [C_TH_300MIL]  143.51,204.47 0 top
C79  .1uF  [C_TH_300MIL]  139.7,80.01 90 top
C80  .1uF  [C_TH_300MIL]  163.83,204.47 0 top
CONN1  HDR_2X25  [HDR_2X25]  130.81,8.89 180 top
CONN2  HDR_2X4  [HDR_2X5]  187.96,8.89 180 top
CONN3  HDR_2X5"  [HDR_2X5']  218.44,53.34 270 top
CONN4  HDR_2X5"  [HDR_2X5']  218.44,20.32 270 top
CONN5  HDR_2X5"  [HDR_2X5']  252.73,53.34 270 top
CONN6  HDR_2X5"  [HDR_2X5']  252.73,20.32 270 top
CONN7  HDR_2X5"  [HDR_2X5']  287.02,53.34 270 top
CONN8  HDR_2X5"  [HDR_2X5']  287.02,20.32 270 top
CONN9  HDR_2X5"  [HDR_2X5']  321.31,53.34 270 top
CONN10  HDR_2X5"  [HDR_2X5']  321.31,20.32 270 top
CONN11  AT_POWER  [AT_POWER]  296.44,6.35 0 top
CONN12  ISA_SLOT8  [ISA_SLOT8]  276.86,210.82 0 top
CONN13  ISA_SLOT8  [ISA_SLOT8]  276.86,190.5 0 top
CONN14  ISA_SLOT8  [ISA_SLOT8]  276.86,170.18 0 top
CONN15  ISA_SLOT8  [ISA_SLOT8]  276.86,149.86 0 top
CONN16  HDR_2X25  [HDR_2X25]  271.78,130.81 180 top
D1  IN5817  [DO35]  134.62,3.81 0 top
D2  IN4148  [DO35]  219.71,210.19 0 top
D3  IN5817  [DO35]  275.59,121.28 0 top
F1  1A  [FUSE]  152.4,3.81 0 top
F2  1A  [FUSE]  289.56,121.28 0 top
J1  HDR_1X3N  [HDR_1X3]  146.69,133.35 270 top
J2  HDR_1X3N  [HDR_1X3]  146.69,110.49 270 top
J3  RESET  [HDR_1X2]  232.41,111.76 270 top
LED1  LED_JUMPER  [LED_JUMPER]  168.91,8.89 270 top
LED2  LED_JUMPER  [LED_JUMPER]  171.45,8.89 270 top
LED3  LED_JUMPER  [LED_JUMPER]  173.99,8.89 270 top
LED4  LED_JUMPER  [LED_JUMPER]  176.53,8.89 270 top
R1  10K  [R_204/7]  219.71,207.01 180 top
R2  100  [R_204/7]  219.71,204.47 0 top
R3  dnf  [R_204/7]  23.5,29.21 90 top
R4  10K  [R_204/7]  146.05,175.26 90 top
R5  10K  [R_204/7]  142.24,175.26 90 top
R6  1K  [R_204/7]  311.15,94.61 0 top
R7  dnf  [R_204/7]  115.57,54.61 90 top
RES1  1K  [RN_SIP6]  2.54,116.2 270 top
RES2  22  [RN_SIP8]  52.07,147.32 0 top
RES3  47  [RN_SIP8]  45.72,80.01 0 top
RES4  47  [RN_SIP8]  45.72,74.93 0 top
RES5  22  [RN_SIP8]  74.93,152.4 0 top
RES6  22  [RN_SIP8]  74.93,147.32 0 top
RES7  22  [RN_SIP8]  68.58,80.01 0 top
RES8  22  [RN_SIP8]  97.79,152.4 0 top
RES9  22  [RN_SIP8]  97.79,147.32 0 top
RES10  47  [RN_SIP8]  91.44,80.01 0 top
RES11  47  [RN_SIP8]  114.3,80.01 0 top
RES12  220/330  [DIL14]  115.57,19.05 180 top
RES13  4.7K  [DIL16]  157.48,67.31 180 top
RES14  220/330  [DIL14]  146.05,19.05 180 top
RES15  220  [RN_SIP8]  184.15,16.51 0 top
RES16  220  [RN_SIP8]  184.15,13.97 0 top
RES17  220/330  [DIL14]  256.54,105.41 180 top
RES18  220/330  [DIL14]  288.29,105.41 180 top
SPARE1  SPARE18  [DIL18]  62.23,191.77 180 top
SPARE2  SPARE20  [DIL20]  39.37,29.21 180 top
SPARE3  SPARE20  [DIL20]  74.93,29.21 180 top
SPARE4  SPARE16  [DIL16]  311.15,119.38 180 top
U1  74LS280  [DIL14]  8.89,160.66 270 top
U2  74LS280  [DIL14]  8.89,137.79 270 top
U3  74LS280  [DIL14]  8.89,114.94 270 top
U4  74LS280  [DIL14]  8.89,92.08 270 top
U5  74AS1004  [DIL14]  41.91,161.29 180 top
U6  SIMM_30  [SIMM_30]  63.5,140.97 0 top
U7  SIMM_30  [SIMM_30]  63.5,133.35 0 top
U8  SIMM_30  [SIMM_30]  63.5,125.73 0 top
U9  SIMM_30  [SIMM_30]  63.5,118.11 0 top
U10  SIMM_30  [SIMM_30]  63.5,110.49 0 top
U11  SIMM_30  [SIMM_30]  63.5,102.87 0 top
U12  SIMM_30  [SIMM_30]  63.5,95.25 0 top
U13  SIMM_30  [SIMM_30]  63.5,87.63 0 top
U14  74AS832  [DIL20]  39.37,67.31 180 top
U15  74AS832  [DIL20]  39.37,54.61 180 top
U16  74AS374  [DIL20_ROUND]  39.37,41.91 180 top
U17  74AS1004  [DIL14]  64.77,161.29 180 top
U18  74AS1034  [DIL14]  66.04,67.31 180 top
U19  22V10  [DIL24]  72.39,54.61 180 top
U20  22V10  [DIL24]  72.39,41.91 180 top
U21  74AS1004  [DIL14]  87.63,173.99 180 top
U22  74AS1004  [DIL14]  87.63,161.29 180 top
U23  74AS1034  [DIL14]  88.9,67.31 180 top
U24  32381  [PGA68]  124.46,184.15 0 top
U25  50 MHz  [DIL14]  127,158.75 180 top
U26  74AS174  [DIL16]  125.73,146.05 180 top
U27  74AS258  [DIL16]  129.54,130.81 180 top
U28  74AS258  [DIL16]  129.54,118.11 180 top
U29  74AS258  [DIL16]  129.54,105.41 180 top
U30  74AS00  [DIL14]  128.27,92.71 180 top
U31  74AS74  [DIL14]  128.27,80.01 180 top
U32  74AS74  [DIL14]  128.27,67.31 180 top
U33  74F138  [DIL16]  129.54,54.61 180 top
U34  20 MHz  [DIL14]  128.27,41.91 180 top
U35  32532  [PGA175]  170.18,168.91 90 top
U36  ALS6311  [DIL20]  162.56,134.62 180 top
U37  16V8  [DIL20_ROUND]  162.56,121.92 180 top
U38  16V8  [DIL20_ROUND]  162.56,106.68 180 top
U39  16V8  [DIL20_ROUND]  162.56,92.71 180 top
U40  16V8  [DIL20_ROUND]  167.64,54.61 180 top
U41  AIC6250  [PLCC68]  171.45,33.02 270 top
U42  74ALS14  [DIL14]  215.9,193.04 180 top
U43  74AS646  [DIL24]  214.63,144.78 180 top
U44  27C256  [DIL28W]  212.09,125.73 180 top
U45  74ALS1034  [DIL14]  213.36,92.71 180 top
U46  32202  [DIL40]  226.06,76.2 180 top
U47  MC145406  [DIL16]  199.39,54.61 180 top
U48  SCN2681  [PLCC44]  201.93,36.83 90 top
U49  MC145406  [DIL16]  199.39,19.05 180 top
U50  74AS174  [DIL16]  240.03,92.71 180 top
U51  MC145406  [DIL16]  233.68,54.61 180 top
U52  SCN2681  [PLCC44]  236.22,36.83 90 top
U53  MC145406  [DIL16]  233.68,19.05 180 top
U54  MC145406  [DIL16]  267.97,54.61 180 top
U55  SCN2681  [PLCC44]  270.51,36.83 90 top
U56  MC145406  [DIL16]  267.97,19.05 180 top
U57  DP8490  [PLCC44']  284.48,82.55 270 top
U58  74AS32  [DIL14]  312.42,105.41 180 top
U59  MC145406  [DIL16]  302.26,54.61 180 top
U60  SCN2681  [PLCC44]  304.8,36.83 90 top
U61  MC145406  [DIL16]  302.26,19.05 180 top
X1  3.6864 MHz  [XTAL]  333.38,36.2 270 top

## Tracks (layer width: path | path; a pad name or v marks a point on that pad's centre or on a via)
1M4M  (via drill 0.33)
  Route2 0.305: U27.3 134.62,133.35 J1.2
  Route15 0.305: v161.29,133.35 163.83,133.35 U36.17
  Bottom 0.305: J1.2 v161.29,133.35
!BANK0
  Top 0.305: U15.2 52.7,53.98 70.48,53.98 U19.19 | U15.5 41.91,59.69 41.91,69.85 U14.5
  Route15 0.305: U15.2 46.99,57.15 41.91,57.15 U15.5 38.1,60.96 35.56,60.96 U14.13
!BANK1
  Route2 0.305: U14.2 U14.19
  Route15 0.305: U14.19 46.99,64.77 41.91,64.77 U14.16 U14.8
  Bottom 0.305: U14.19 50.8,60.96 55.24,60.96 56.52,59.69 56.52,58.42 57.78,57.15 59.69,57.15 U19.16
!BCLK  (via drill 0.33)
  Top 0.305: v120.65,93.34 122.56,91.44 125.73,91.44 127,90.17 127,87.63 U31.3 | U35.C8 154.94,166.37 154.94,161.93 154.31,161.29 145.41,161.29 C23.1
  Route2 0.305: U32.11 132.08,67.31 132.08,72.39 129.54,74.93 129.54,81.28 130.81,82.55 U31.3 | v120.65,93.34 118.75,95.25 118.75,140.34 | 118.75,140.34 U26.9 | 118.75,140.34 130.18,140.34 130.81,140.97 130.81,143.51 135.89,148.59 135.89,158.12 C23.1
  Route15 0.305: R7.2 116.2,58.42 118.11,60.33 125.09,60.33 U32.11
!BCLK_CLR
  Top 0.305: U30.8 124.46,85.09 124.46,82.55 126.36,80.64 128.27,80.64 132.08,76.83 132.08,74.93 U32.1
  Route2 0.305: U32.13 135.89,66.04 U32.1
!BE0
  Route2 0.305: U35.S12 187.96,176.53 177.8,176.53 170.18,168.91 128.91,168.91 123.19,163.19 123.19,151.13 U26.6
!BE0L
  Top 0.305: U19.1 88.9,60.96 101.6,60.96 102.87,62.23 102.87,130.81 119.38,147.32 U26.7
  Route15 0.305: U16.18 45.72,41.27 49.53,45.09 49.53,46.99 52.7,50.16 52.7,51.44 54.61,53.34 81.28,53.34 U19.1
!BE0LP
  Route15 0.305: U20.5 71.75,41.27 51.44,41.27 U16.19
!BE1
  Top 0.305: U35.P10 182.88,171.45 175.26,171.45 160.02,156.21 148.59,156.21 146.05,153.67 128.27,153.67 125.73,151.13 125.73,146.05 U26.11
!BE1L
  Top 0.305: U26.10 118.11,140.97 114.3,140.97 107.95,134.62 107.95,62.23 102.87,57.15 85.09,57.15 U19.2
  Route15 0.305: U16.3 49.53,49.53 49.53,52.07 52.07,54.61 80.01,54.61 U19.2
!BE1LP
  Route2 0.305: U16.2 50.16,43.81 59.05,43.81 U20.11
!BE2
  Route2 0.305: U26.13 128.27,143.51 128.27,156.21 133.35,161.29 133.35,163.83 135.89,166.37 170.18,166.37 177.8,173.99 187.96,173.99 U35.S11
!BE2L
  Top 0.305: U19.3 83.82,55.88 104.14,55.88 110.49,62.23 110.49,83.19 111.76,84.45 111.76,133.35 118.11,139.7 121.92,139.7 U26.12
  Route15 0.305: U16.17 43.18,43.18 44.45,44.45 44.45,46.99 46.99,49.53 46.99,51.44 51.44,55.88 78.74,55.88 U19.3
!BE2LP
  Route2 0.305: U16.16 43.81,41.27 57.78,41.27 U20.14
!BE3
  Top 0.305: U26.14 132.08,144.78 139.7,144.78 148.59,153.67 161.93,153.67 162.56,154.31 162.56,156.21 175.26,168.91 184.78,168.91 185.42,169.54 185.42,171.45 U35.R10
!BE3L  (via drill 0.33)
  Top 0.305: U26.15 127,137.16 120.65,137.16 115.57,132.08 v115.57,69.85
  Route15 0.305: U16.4 43.18,47.62 44.45,48.9 44.45,52.07 49.53,57.15 77.47,57.15 U19.4
  Bottom 0.305: v115.57,69.85 106.68,60.96 81.28,60.96 U19.4
!BE3LP
  Route2 0.305: U16.5 43.81,42.55 60.33,42.55 U20.10
!BMT  (via drill 0.33)
  Top 0.305: v147.96,81.92 151.76,81.92 157.48,87.63 157.48,93.34 158.75,94.61 U39.7 | U38.4 170.18,114.3 v181.61,114.3
  Route2 0.305: v181.61,114.3 182.88,114.3 193.04,124.46 193.04,139.06 194.94,140.97 194.94,176.53 191.13,180.34 U35.S13
  Bottom 0.305: U19.6 77.47,62.23 104.14,62.23 120.65,78.74 144.78,78.74 v147.96,81.92 | U39.7 162.56,100.33 162.56,104.14 166.37,107.95 U38.4
!BOUT  (via drill 0.33)
  Route2 0.305: v167.64,127.64 170.18,130.18 170.18,139.06 170.81,139.7 190.5,139.7 191.77,140.97 191.77,167.64 U35.S9
  Bottom 0.305: U39.6 165.1,100.33 166.37,100.33 167.64,101.6 v167.64,127.64
!CAS
  Bottom 0.305: U19.7 72.39,59.69 72.39,64.77 74.93,67.31 107.95,67.31 118.75,78.11 118.75,84.45 U30.9 124.46,87.63 146.05,87.63 149.22,90.81 154.31,90.81 U39.13
!CAS0
  Route2 0.305: U19.15 67.31,54.61 67.31,68.58 68.58,69.85 U18.3
  Route15 0.305: U18.3 75.56,64.14 75.56,62.87 76.2,62.23 92.71,62.23 U23.13
!CAS1
  Route2 0.305: U18.1 69.85,67.31 69.85,54.61 68.58,53.34 U19.17
  Route15 0.305: U23.1 95.25,72.39 74.93,72.39 U18.1
!CAS2
  Route2 0.305: U19.18 77.47,57.15 77.47,59.69 80.01,62.23 80.01,64.77 U23.5
  Route15 0.305: U23.11 86.36,66.04 U23.5
!CAS3
  Route2 0.305: U19.22 81.28,55.88 80.01,57.15 80.01,59.69 U23.9 U23.3
!CASA0
  Route2 0.305: U18.4 71.12,76.2 72.39,76.2 RES10.7
!CASA0R
  Top 0.305: U6.28 34.29,143.51 95.25,143.51 U6.2 97.79,139.7 93.98,135.89 93.98,132.08 88.9,127 88.9,124.46 83.82,119.38 83.82,116.84 78.74,111.76 78.74,85.09 RES10.8
!CASA1
  Route2 0.305: U18.2 74.93,74.93 76.2,74.93 RES10.5
!CASA1R
  Top 0.305: RES10.6 83.82,85.09 83.82,104.14 88.9,109.22 88.9,111.76 93.98,116.84 93.98,121.92 U8.2
  Bottom 0.305: U8.28 33.66,123.83 95.89,123.83 U8.2
!CASA2
  Route2 0.305: U23.6 86.36,73.66 RES10.3
!CASA2R
  Top 0.305: U10.2 91.44,104.14 91.44,92.71 88.9,90.17 88.9,85.09 RES10.4
  Bottom 0.305: U10.2 95.89,108.58 33.66,108.58 U10.28
!CASA3
  Route2 0.305: RES10.1 87.63,76.2 87.63,69.85 U23.8
!CASA3R
  Route2 0.305: RES10.2 91.44,82.55 92.71,82.55 96.52,86.36 96.52,93.98 U12.2
  Bottom 0.305: U12.2 95.89,93.34 33.66,93.34 U12.28
!CASB0
  Route2 0.305: RES11.1 101.6,67.31 95.25,67.31 U23.12
!CASB0R
  Route2 0.305: RES11.2 104.14,87.63 104.14,127 U7.2
  Bottom 0.305: U7.28 33.66,135.25 95.89,135.25 U7.2
!CASB1
  Route2 0.305: RES11.3 104.14,74.93 97.79,74.93 U23.2
!CASB1R
  Route2 0.305: RES11.4 102.87,83.82 102.87,113.03 U9.2
  Bottom 0.305: U9.2 95.89,120.02 33.66,120.02 U9.28
!CASB2
  Route2 0.305: RES11.5 100.33,76.2 96.52,76.2 92.71,72.39 92.71,69.85 U23.10
!CASB2R
  Route2 0.305: RES11.6 99.06,82.55 99.06,101.6 U11.2
  Bottom 0.305: U11.28 33.66,100.97 95.89,100.97 U11.2
!CASB3
  Route2 0.305: U23.4 95.25,77.47 96.52,77.47 RES11.7
!CASB3R
  Route2 0.305: RES11.8 97.79,81.28 U13.2
  Bottom 0.305: U13.2 95.89,85.72 33.66,85.72 U13.28
!CASP
  Top 0.305: U20.2 85.09,46.99 159.38,46.99 162.56,50.16 162.56,52.07 167.64,57.15 167.64,87.63 U39.18
!CONF  (via drill 0.33)
  Top 0.305: v158.75,76.83 157.48,76.83 154.94,74.3 154.94,52.07 U40.11 154.94,49.53 v107.31,49.53 | v213.36,99.06 224.16,109.86 224.16,112.39 226.06,114.3 227.33,114.3 229.87,116.84 229.87,141.6 224.79,146.69 224.79,150.5 v221.62,153.67
  Route2 0.305: v152.4,106.05 152.4,124.46 U37.9
  Route15 0.305: v158.75,76.83 165.1,83.19 165.1,92.08 162.56,94.61 162.56,99.06 | 162.56,99.06 156.21,99.06 154.94,100.33 154.94,103.5 v152.4,106.05 | 162.56,99.06 166.37,99.06 U39.3 171.45,99.06 v213.36,99.06 | U35.N10 182.88,171.45 190.5,171.45 208.28,153.67 v221.62,153.67
  Bottom 0.305: U19.13 58.42,50.16 61.59,46.99 104.78,46.99 v107.31,49.53
!CTS0
  Top 0.305: U47.13 199.39,49.53 199.39,34.29 U48.8
!CTS1
  Route2 0.305: U49.13 199.39,16.51 199.39,31.75 198.12,33.02 U48.5
!CTS2
  Top 0.305: U52.8 233.68,34.29 233.68,49.53 U51.13
!CTS3
  Route2 0.305: U52.5 231.14,31.75 231.14,19.05 U53.13
!CTS4
  Top 0.305: U54.13 267.97,49.53 267.97,34.29 U55.8
!CTS5
  Route2 0.305: U55.5 265.43,31.75 265.43,19.05 U56.13
!CTS6
  Top 0.305: U60.8 302.26,34.29 302.26,49.53 U59.13
!CTS7
  Route2 0.305: U60.5 299.72,31.75 299.72,19.05 U61.13
!DACK
  Top 0.305: U40.6 164.47,56.52 161.29,56.52 160.02,57.78 160.02,97.79 158.12,99.69 155.57,99.69 153.67,101.6 U38.12
!DACK0
  Route15 0.305: U40.17 170.18,49.53 170.18,44.45 U41.19
!DACK1  (via drill 0.33)
  Route2 0.305: U57.29 275.59,71.12 v275.59,62.23 | U40.16 170.18,49.53 179.71,49.53 180.34,50.16 180.34,50.8 v187.96,58.42
  Bottom 0.305: v275.59,62.23 274.32,60.96 190.5,60.96 v187.96,58.42
!DCD0
  Top 0.305: U47.11 196.85,49.53 196.85,36.83 U48.3
!DCD1
  Top 0.305: U48.40 191.77,41.91 191.77,19.05 U49.11
!DCD2
  Top 0.305: U51.11 231.14,49.53 231.14,36.83 U52.3
!DCD3
  Top 0.305: U52.40 226.06,41.91 226.06,19.05 U53.11
!DCD4
  Top 0.305: U54.11 265.43,49.53 265.43,36.83 U55.3
!DCD5
  Top 0.305: U56.11 260.35,19.05 260.35,41.91 U55.40
!DCD6
  Top 0.305: U59.11 299.72,49.53 299.72,36.83 U60.3
!DCD7
  Top 0.305: U60.40 294.64,41.91 294.64,19.05 U61.11
!DDIN  (via drill 0.33)
  Top 0.305: U39.8 144.78,85.09 v144.78,84.45 143.51,85.72 133.99,85.72 U30.12 | v149.22,115.57 150.5,114.3 160.02,114.3 U38.5
  Route2 0.305: U19.14 62.87,48.9 103.5,48.9 106.68,52.07 110.49,52.07 114.3,55.88 142.88,55.88 144.78,57.78 v144.78,84.45
  Route15 0.305: v146.69,142.88 146.69,139.06 145.41,137.79 145.41,119.38 v149.22,115.57
  Bottom 0.305: U39.8 160.02,100.33 160.02,106.05 163.83,109.86 U38.5 | v146.69,142.88 144.78,144.78 134.62,144.78 U26.3 125.73,153.67 125.73,170.18 U24.L6 125.73,172.72 125.73,175.26 128.27,177.8 148.59,177.8 149.86,176.53 177.8,176.53 180.34,173.99 187.96,173.99 U35.S10
!DDINL  (via drill 0.33)
  Top 0.305: U30.13 127,95.25 119.38,95.25 118.11,93.98 118.11,68.58 116.84,67.31 113.03,67.31 | 113.03,67.31 113.03,132.08 119.38,138.43 123.19,138.43 125.73,140.97 125.73,143.51 U26.2 | 113.03,67.31 113.03,62.23 103.5,52.7 85.72,52.7 U19.23
  Route15 0.305: U43.3 222.25,147.32 222.25,132.08 214.63,124.46 200.66,124.46 184.15,140.97 173.99,140.97 v172.72,142.24
  Bottom 0.305: v172.72,142.24 172.72,155.57 172.09,156.21 148.59,156.21 139.7,147.32 134.62,147.32 U26.2
!DRAM  (via drill 0.33)
  Top 0.305: U15.18 48.26,48.26 155.57,48.26 157.48,50.16 157.48,73.66 v158.12,74.3 | U37.15 162.56,116.84 v182.88,116.84
  Route2 0.305: U35.P13 185.42,179.07 190.5,179.07 193.68,175.9 193.68,140.97 191.77,139.06 191.77,125.73 v182.88,116.84 | v158.12,74.3 160.02,74.3 170.18,84.45 170.18,95.25 U39.2 170.18,97.79 170.18,114.3 168.91,115.57 163.83,115.57 U37.15
!DTR0
  Top 0.305: U47.12 199.39,52.07 203.84,52.07 204.47,51.44 204.47,46.99 U48.31
!DTR1
  Route2 0.305: U48.15 207.01,26.67 207.01,14.61 206.38,13.97 199.39,13.97 U49.12
!DTR2
  Top 0.305: U52.31 238.76,46.99 238.76,51.44 238.12,52.07 233.68,52.07 U51.12
!DTR3
  Route2 0.305: U52.15 241.3,26.67 241.3,14.61 240.66,13.97 233.68,13.97 U53.12
!DTR4
  Top 0.305: U55.31 273.05,46.99 273.05,51.44 272.42,52.07 267.97,52.07 U54.12
!DTR5
  Route2 0.305: U55.15 275.59,26.67 275.59,14.61 274.95,13.97 267.97,13.97 U56.12
!DTR6
  Top 0.305: U60.31 307.34,46.99 307.34,51.44 306.7,52.07 302.26,52.07 U59.12
!DTR7
  Route2 0.305: U60.15 309.88,26.67 309.88,14.61 309.25,13.97 302.26,13.97 U61.12
!DUA0  (via drill 0.33)
  Top 0.305: U46.39 246.38,67.31 243.84,64.77 v232.41,64.77
  Route2 0.305: v232.41,64.77 231.14,63.5 218.44,63.5 v217.17,62.23 218.44,60.96 218.44,45.72 U48.24
  Route15 0.305: RES13.11 156.21,60.96 v182.88,60.96
  Bottom 0.305: v182.88,60.96 186.69,60.96 187.96,62.23 v217.17,62.23
!DUA1
  Route2 0.305: U52.24 246.38,39.37 246.38,45.72 245.11,46.99 245.11,67.31 U46.38
  Route15 0.305: RES13.13 161.29,66.04 241.3,66.04 U46.38
!DUA2
  Route2 0.305: U55.24 278.13,36.83 260.99,36.83 257.18,40.64 257.18,62.87 250.19,69.85 242.57,69.85 U46.37
  Route15 0.305: U46.37 242.57,69.85 244.47,69.85 245.11,69.22 245.11,67.31 242.57,64.77 238.76,64.77 237.49,63.5 227.97,63.5 226.69,64.77 162.56,64.77 RES13.14
!DUA3
  Bottom 0.305: RES13.6 154.94,69.85 237.49,69.85 U46.36 241.3,66.04 283.21,66.04 290.19,59.05 290.19,56.52 294.64,52.07 294.64,49.53 296.55,47.62 311.79,47.62 314.96,44.45 314.96,39.37 U60.24
!DUAR0
  Top 0.305: U48.30 205.74,40.64 U48.16
  Route2 0.305: U46.5 237.49,85.09 235.59,85.09 234.95,84.45 234.95,77.47 227.33,69.85 227.33,67.31 226.06,66.04 218.44,66.04 215.9,63.5 215.9,44.45 213.36,41.91 209.55,41.91 U48.30 207.01,41.91 190.5,41.91 185.42,46.99 156.21,46.99 149.86,53.34 149.86,69.85 RES13.7
!DUAR1  (via drill 0.33)
  Top 0.305: U52.16 240.03,40.64 U52.30
  Route2 0.305: U52.30 241.3,44.45 241.3,60.96 v240.03,62.23 240.03,80.01 U46.6
  Route15 0.305: RES13.15 165.1,62.23 190.5,62.23 191.77,63.5 226.06,63.5 227.33,62.23 v240.03,62.23
!DUAR2
  Top 0.305: U55.30 274.32,40.64 U55.16
  Route2 0.305: U55.30 275.59,44.45 275.59,46.99 273.05,49.53 273.05,51.44 267.97,56.52 267.97,59.69 250.19,77.47 245.11,77.47 240.03,82.55 240.03,85.09 238.76,86.36 234.95,86.36 233.68,85.09 U46.7
  Route15 0.305: RES13.9 154.94,69.85 189.87,69.85 196.22,76.2 208.28,76.2 213.36,81.28 225.43,81.28 227.33,83.19 227.33,84.45 227.97,85.09 232.41,85.09 U46.7
!DUAR3  (via drill 0.33)
  Top 0.305: U60.16 308.61,40.64 U60.30
  Route15 0.305: U46.8 227.33,80.01 214.63,80.01 209.55,74.93 196.85,74.93 190.5,68.58 156.21,68.58 RES13.10 | v266.7,81.28 267.97,80.01 279.4,80.01 281.94,77.47 281.94,73.03 292.74,62.23 309.88,62.23 312.42,59.69 312.42,44.45 U60.30
  Bottom 0.305: U46.8 233.68,81.28 v266.7,81.28
!DUART  (via drill 0.33)
  Route2 0.305: U33.4 133.35,60.96 140.34,60.96 142.88,63.5 v142.88,95.89
  Route15 0.305: v142.88,95.89 142.88,99.06 151.76,107.95 153.67,107.95 154.94,109.22 154.94,111.76 160.02,116.84 160.02,118.75 160.66,119.38 167.64,119.38 U37.18
!DUART0
  Bottom 0.305: U33.15 137.16,52.07 185.42,52.07 191.77,45.72 U48.39
!DUART1
  Bottom 0.305: U52.39 228.6,46.99 191.77,46.99 185.42,53.34 135.89,53.34 U33.14
!DUART2
  Bottom 0.305: U33.13 134.62,54.61 185.42,54.61 187.96,52.07 247.65,52.07 250.19,49.53 256.54,49.53 260.35,45.72 U55.39
!DUART3
  Bottom 0.305: U60.39 295.91,45.72 289.56,52.07 250.19,52.07 247.65,54.61 186.69,54.61 185.42,55.88 133.35,55.88 U33.12
!EOP  (via drill 0.33)
  Top 0.305: U38.19 175.26,99.06 182.25,99.06 207.01,74.3 v213.36,74.3 | U57.30 276.86,77.47 243.84,77.47 240.66,80.64 v230.5,80.64
  Route15 0.305: v213.36,74.3 217.81,78.74 228.6,78.74 v230.5,80.64
!EPROM
  Route2 0.305: U37.14 158.75,120.02 159.38,120.65 170.18,120.65 170.18,116.84 171.45,115.57 U38.2
  Route15 0.305: U38.2 173.99,113.03 203.2,113.03 U44.20
!FFSR
  Top 0.305: U35.B6 152.4,163.83 152.4,165.74 151.76,166.37 150.5,166.37 149.86,167 149.86,168.28 148.59,169.54 144.15,169.54 R5.1
  Route2 0.305: R5.1 U24.L10
!HSA  (via drill 0.33)
  Top 0.305: U15.19 49.53,49.53 102.87,49.53 109.22,55.88 146.05,55.88 152.4,62.23 152.4,73.66 158.12,79.38 v158.75,79.38
  Route2 0.305: v158.75,79.38 159.38,79.38 167.64,87.63 167.64,95.25 U39.4
  Bottom 0.305: U39.4 170.18,100.33 170.18,128.27 168.91,129.54 U36.18
!HSAC
  Bottom 0.305: U50.7 229.87,100.33 175.26,100.33 172.72,97.79 172.72,95.89 170.18,93.34 131.44,93.34 U30.4
!HSADR
  Route2 0.305: U19.11 57.78,55.24 47.62,55.24 U15.17
!ICU  (via drill 0.33)
  Route2 0.305: U46.21 199.39,69.85 v199.39,101.6
  Route15 0.305: v199.39,101.6 163.19,101.6 162.56,102.23 162.56,106.68 160.02,109.22 160.02,113.03 162.56,115.57 163.83,115.57 U37.17
!INT  (via drill 0.33)
  Route2 0.305: U35.B7 154.94,163.83 184.78,163.83 185.42,163.19 v185.42,146.05
  Bottom 0.305: U46.2 247.65,85.09 247.65,97.79 238.12,107.31 222.88,107.31 219.71,110.49 219.71,120.02 212.72,127 196.85,127 185.42,138.43 v185.42,146.05
!INT15
  Route15 0.305: U46.1 246.38,86.36 211.46,86.36 209.55,84.45 209.55,82.55 204.47,77.47 195.58,77.47 189.23,71.12 173.99,71.12 172.72,72.39 167.64,72.39 RES13.1
!IODEC
  Route15 0.305: U35.S15 187.96,184.15 180.97,184.15 180.34,183.51 180.34,181.61 170.18,171.45 170.18,168.91 162.56,161.29 150.5,161.29 149.86,160.66 149.86,121.92 U37.12
!IOINH
  Bottom 0.305: U37.8 157.48,127 160.66,127 162.56,128.91 162.56,139.7 161.29,140.97 U35.E1
!IR1
  Top 0.305: U46.33 231.14,74.93 224.79,81.28 224.79,85.09 227.33,87.63 236.85,87.63 237.49,88.27 237.49,104.14 260.35,127 260.35,133.99 266.7,140.34 273.69,140.34 278.13,144.78 284.48,144.78 CONN15.A13
  Bottom 0.305: CONN15.A13 287.02,149.86 285.75,151.13 285.75,163.83 287.02,165.1 CONN14.A13 287.02,170.18 285.75,171.45 285.75,184.15 287.02,185.42 CONN13.A13 287.02,190.5 285.75,191.77 285.75,204.47 287.02,205.74 CONN12.A13
!IR2
  Top 0.305: CONN15.A12 285.12,142.88 278.76,142.88 274.32,138.43 267.33,138.43 262.89,133.99 262.89,127 240.03,104.14 240.03,87.63 238.76,86.36 228.6,86.36 U46.10
  Bottom 0.305: CONN15.A12 289.56,149.86 288.29,151.13 288.29,163.83 289.56,165.1 CONN14.A12 289.56,170.18 288.29,171.45 288.29,184.15 289.56,185.42 CONN13.A12 289.56,190.5 288.29,191.77 288.29,204.47 289.56,205.74 CONN12.A12
!IR3
  Top 0.305: CONN15.A11 289.56,149.86 276.86,149.86 275.59,148.59 275.59,145.41 272.42,142.24 266.06,142.24 257.81,133.99 257.81,127 234.95,104.14 234.95,95.25 229.87,90.17 227.97,90.17 222.25,84.45 222.25,81.28 229.87,73.66 229.87,67.94 230.5,67.31 232.41,67.31 U46.34
  Bottom 0.305: CONN15.A11 292.1,149.86 290.83,151.13 290.83,163.83 292.1,165.1 CONN14.A11 292.1,170.18 290.83,171.45 290.83,184.15 292.1,185.42 CONN13.A11 292.1,190.5 290.83,191.77 290.83,204.47 292.1,205.74 CONN12.A11
!NMI  (via drill 0.33)
  Route2 0.305: U20.17 74.3,43.81 92.71,43.81 96.52,47.62 109.22,47.62 116.2,54.61 144.15,54.61 147.32,57.78 147.32,78.11 149.86,80.64 149.86,113.67 151.13,114.94 v151.13,116.2
  Route15 0.305: RES1.5 3.81,111.12 3.81,77.47 27.94,53.34 34.92,53.34 36.83,51.44 36.83,48.9 39.37,46.35 39.37,45.09 41.91,42.55 41.91,37.47 42.55,36.83 67.31,36.83 U20.17 | v151.13,116.2 148.59,118.75 148.59,162.56 U35.A7
!NRDY  (via drill 0.33)
  Top 0.305: U30.1 137.79,98.42 144.15,98.42 150.5,104.78 154.31,104.78 U38.13 158.75,105.41 173.35,105.41 173.99,104.78 v185.42,104.78
  Route15 0.305: v185.42,104.78 186.69,103.5 236.85,103.5 U50.3
!NRDYR
  Route15 0.305: U39.16 158.75,93.98 135.89,93.98 U30.2
!PARCLU
  Bottom 0.305: U33.10 121.92,52.07 111.12,52.07 109.86,50.8 106.05,50.8 103.5,48.26 61.59,48.26 59.69,50.16 59.69,51.44 58.42,52.7 42.55,52.7 U15.16
!PARITYC
  Route2 0.305: U15.14 38.73,47.62 71.75,47.62 U20.6
!PARITYR
  Top 0.305: U15.11 29.21,49.53 29.21,45.09 31.75,42.55 53.98,42.55 U20.13
!PARRDU
  Bottom 0.305: U15.13 36.2,53.98 60.33,53.98 62.23,52.07 62.23,50.16 62.87,49.53 101.6,49.53 104.14,52.07 107.95,52.07 109.22,53.34 123.19,53.34 U33.11
!PERG  (via drill 0.33)
  Route15 0.305: U58.6 304.17,112.39 299.08,112.39 296.55,114.94 253.37,114.94 239.4,128.91 v239.4,144.15
  Bottom 0.305: v239.4,144.15 232.41,151.13 219.71,151.13 | 219.71,151.13 218.44,151.13 190.5,179.07 187.96,179.07 U35.R13 | 219.71,151.13 219.71,142.24 U43.21
!RAS  (via drill 0.33)
  Top 0.305: U15.1 53.34,55.88 71.12,55.88 U19.20
  Route2 0.305: U14.7 35.56,68.58 U14.12 31.75,62.23 36.83,62.23 U14.15 | U14.18 45.72,60.96 U15.4 | U14.1 52.07,69.85 52.07,59.69 U15.1 49.53,57.15 44.45,57.15 U15.4 | U14.4 41.91,69.85 41.91,59.69 U15.4
  Route15 0.305: U14.7 36.83,69.85 41.91,69.85 U14.4 | U14.1 57.15,77.47 127,77.47 U31.2 | v171.45,92.08 v180.97,92.08
  Bottom 0.305: U31.2 135.89,86.36 151.13,86.36 U39.12 155.57,87 158.75,87 160.02,88.27 160.02,90.17 161.93,92.08 v171.45,92.08 | U50.6 234.31,94.61 228.6,94.61 224.79,98.42 217.81,98.42 217.17,97.79 217.17,95.89 215.26,93.98 205.1,93.98 203.2,92.08 v180.97,92.08
!RASA0
  Route2 0.305: RES3.7 30.48,77.47 29.21,76.2 29.21,64.77 U14.11
!RASA0R
  Route2 0.305: RES3.8 27.94,134.62 U6.27
!RASA1
  Route2 0.305: RES3.5 39.37,76.2 39.37,73.66 38.1,72.39 U14.6
!RASA1R
  Route2 0.305: RES3.6 33.02,124.46 U8.27
!RASA2
  Route2 0.305: U15.3 46.99,59.69 46.99,78.74 RES3.1
!RASA2R
  Route15 0.305: RES3.2 38.1,85.09 38.1,106.68 U10.27
!RASA3
  Route2 0.305: U15.6 39.37,59.69 39.37,72.39 40.64,73.66 RES4.3
!RASA3R
  Route15 0.305: RES4.4 34.29,78.74 34.29,81.28 33.02,82.55 33.02,93.98 U12.27
!RASB0
  Route2 0.305: RES4.7 U14.9
!RASB0R
  Route2 0.305: RES4.8 27.94,76.2 29.21,77.47 29.21,85.09 30.48,86.36 30.48,129.54 U7.27
!RASB1
  Route2 0.305: RES4.5 36.83,73.66 36.83,64.77 U14.14
!RASB1R
  Route2 0.305: U9.27 35.56,116.84 35.56,82.55 34.29,81.28 34.29,76.2 RES4.6
!RASB2
  Route2 0.305: RES4.1 U14.3
!RASB2R
  Route15 0.305: RES4.2 39.37,78.74 39.37,81.28 35.56,85.09 35.56,101.6 U11.27
!RASB3
  Route2 0.305: RES3.3 44.45,76.2 44.45,64.77 U14.17
!RASB3R
  Route15 0.305: RES3.4 34.29,83.82 U13.27
!RD
  Top 0.305: U52.10 231.14,29.21 229.24,29.21 228.6,29.84 228.6,44.45 223.52,49.53 U46.30
  Route2 0.305: U46.30 222.25,67.31 212.72,67.31 212.09,67.94 212.09,90.17 214.63,92.71 214.63,101.6 213.36,102.87 U44.22 213.36,129.54 212.09,130.81 212.09,134.62 214.63,137.16 222.25,137.16 U43.23
  Route15 0.305: U60.10 299.72,29.21 267.97,29.21 U55.10 265.43,29.21 233.68,29.21 U52.10 231.14,29.21 199.39,29.21 U48.10 196.85,29.21 194.31,29.21 186.69,21.59 180.34,21.59 U41.58 | U46.30 231.14,76.2 273.05,76.2 274.32,77.47 276.86,77.47 U57.27 | U38.17 166.37,103.5 171.45,108.58 203.84,108.58 U44.22
  Bottom 0.305: U15.15 36.2,48.9 32.38,48.9 U15.12 29.21,49.53 29.21,37.47 30.48,36.2 152.4,36.2 155.57,39.37 161.93,39.37 177.8,23.5 177.8,21.59 U41.58
!RDY  (via drill 0.33)
  Route2 0.305: U30.3 132.72,98.42 139.06,98.42 140.34,99.69 140.34,114.94 148.59,123.19 v151.13,123.19
  Route15 0.305: v151.13,123.19 152.4,124.46 152.4,158.12 153.03,158.75 161.29,158.75 177.8,175.26 U35.N11
!RFCYL
  Route2 0.305: U39.14 157.48,90.17 157.48,121.92 160.02,124.46 160.02,127 U36.16
  Route15 0.305: U19.5 78.74,60.96 101.6,60.96 114.3,73.66 143.51,73.66 U39.14
!RFRQI
  Bottom 0.305: U19.21 81.28,53.34 106.68,53.34 109.22,55.88 116.2,55.88 120.65,60.33 122.56,60.33 124.46,62.23 124.46,64.77 129.54,69.85 129.54,73.03 130.81,74.3 143.51,74.3 154.94,85.72 159.38,85.72 161.29,87.63 U39.15
!RSTO  (via drill 0.33)
  Top 0.305: U35.A6 148.59,162.56 147.96,163.19 147.96,167 v147.32,167.64 | U57.31 279.4,74.93 279.4,84.45 278.76,85.09 274.32,85.09 268.61,90.81 248.28,90.81 U50.15 | U20.3 82.55,44.45 162.56,44.45 U41.24 165.1,44.45 165.1,42.55 166.37,41.27 172.09,41.27 172.72,41.91 172.72,46.99 174.62,48.9 179.07,48.9 180.34,50.16 180.34,53.34 184.78,57.78 184.78,59.05 196.22,70.48 214,70.48 U46.27
  Route2 0.305: U24.A9 134.62,199.39 160.02,199.39 167.64,207.01 184.15,207.01 234.95,156.21 234.95,113.03 237.49,110.49 237.49,93.98 | 237.49,93.98 241.3,93.98 U50.15 | 237.49,93.98 227.97,93.98 226.69,92.71 226.69,88.9 222.25,84.45 222.25,78.74 219.07,75.56 219.07,71.75 U46.27
  Route15 0.305: v147.32,167.64 147.32,190.5 135.89,201.93 132.72,201.93 132.08,201.29 U24.A9
!RSTOUS  (via drill 0.33)
  Route15 0.305: v234.95,106.05 234.95,109.22 236.22,110.49 236.22,154.94 232.41,158.75 232.41,177.8 222.25,187.96 222.25,190.5 U42.4
  Bottom 0.305: U50.14 242.57,90.17 242.57,97.79 234.95,105.41 v234.95,106.05
!RTS0
  Route2 0.305: U48.32 204.47,44.45 204.47,46.99 203.2,48.26 195.58,48.26 U47.10
!RTS1
  Route2 0.305: U49.10 195.58,12.7 208.28,12.7 209.55,13.97 209.55,31.11 208.91,31.75 204.47,31.75 U48.14
!RTS2
  Route2 0.305: U52.32 238.76,44.45 238.76,46.99 237.49,48.26 229.87,48.26 U51.10
!RTS3
  Route2 0.305: U53.10 229.87,12.7 242.57,12.7 243.84,13.97 243.84,31.11 243.21,31.75 238.76,31.75 U52.14
!RTS4
  Route2 0.305: U55.32 273.05,44.45 273.05,46.99 271.78,48.26 264.16,48.26 U54.10
!RTS5
  Route2 0.305: U56.10 264.16,12.7 276.86,12.7 278.13,13.97 278.13,31.11 277.5,31.75 273.05,31.75 U55.14
!RTS6
  Route15 0.305: U59.10 298.45,48.26 306.07,48.26 307.34,46.99 307.34,44.45 U60.32
!RTS7
  Route2 0.305: U61.10 298.45,12.7 311.15,12.7 312.42,13.97 312.42,31.11 311.79,31.75 307.34,31.75 U60.14
!RXD0
  Top 0.305: U48.35 201.93,44.45 206.38,44.45 207.01,45.09 207.01,49.53 U47.15
!RXD1
  Route2 0.305: U48.11 201.93,29.21 203.84,29.21 204.47,28.57 204.47,16.51 U49.15
!RXD2
  Top 0.305: U51.15 241.3,49.53 241.3,45.09 240.66,44.45 236.22,44.45 U52.35
!RXD3
  Route2 0.305: U52.11 236.22,29.21 238.12,29.21 238.76,28.57 238.76,16.51 U53.15
!RXD4
  Top 0.305: U54.15 275.59,49.53 275.59,45.09 274.95,44.45 270.51,44.45 U55.35
!RXD5
  Route2 0.305: U55.11 270.51,29.21 272.42,29.21 273.05,28.57 273.05,16.51 U56.15
!RXD6
  Top 0.305: U60.35 304.8,44.45 309.25,44.45 309.88,45.09 309.88,49.53 U59.15
!RXD7
  Route2 0.305: U60.11 304.8,29.21 306.7,29.21 307.34,28.57 307.34,16.51 U61.15
!SACK
  Bottom 0.305: U57.16 279.4,90.17 279.4,100.33 RES18.8 278.13,101.6 256.54,123.19 CONN16.38 255.27,130.81 255.27,142.24 256.54,143.51 CONN15.A25 256.54,149.86 255.27,151.13 255.27,163.83 256.54,165.1 CONN14.A25 256.54,170.18 255.27,171.45 255.27,184.15 256.54,185.42 CONN13.A25 256.54,190.5 255.27,191.77 255.27,204.47 256.54,205.74 CONN12.A25
!SACK0
  Route2 0.305: RES12.12 144.78,41.91 160.02,41.91 U41.28
  Bottom 0.305: CONN1.38 116.84,8.89 116.84,12.06 118.11,13.34 RES12.12
!SATN
  Route2 0.305: RES18.10 285.75,99.06 U57.17
  Bottom 0.305: RES18.10 283.21,104.14 279.4,104.14 264.16,119.38 CONN16.32 262.89,130.81 262.89,142.88 261.62,144.15 CONN15.A23 261.62,149.86 260.35,151.13 260.35,163.83 261.62,165.1 CONN14.A23 261.62,170.18 260.35,171.45 260.35,184.15 261.62,185.42 CONN13.A23 261.62,190.5 260.35,191.77 260.35,204.47 261.62,205.74 CONN12.A23
!SATN0
  Bottom 0.305: CONN1.32 124.46,8.89 124.46,11.43 133.35,20.32 139.06,20.32 140.97,22.23 RES14.6 148.59,30.48 156.21,30.48 U41.35
!SBSY
  Bottom 0.305: U57.15 280.67,99.06 RES18.9 281.94,102.87 278.76,102.87 259.08,122.56 CONN16.36 257.81,130.81 257.81,142.24 259.08,143.51 CONN15.A24 259.08,149.86 257.81,151.13 257.81,163.83 259.08,165.1 CONN14.A24 259.08,170.18 257.81,171.45 257.81,184.15 259.08,185.42 CONN13.A24 259.08,190.5 257.81,191.77 257.81,204.47 259.08,205.74 CONN12.A24
!SBSY0
  Route2 0.305: RES12.13 142.24,36.83 152.4,36.83 154.94,39.37 160.02,39.37 U41.30
  Bottom 0.305: CONN1.36 119.38,8.89 119.38,12.06 120.65,13.34 RES12.13
!SCD
  Bottom 0.305: U57.20 274.32,86.36 271.78,88.9 271.78,96.52 262.89,105.41 260.35,105.41 RES17.4 246.38,119.38 CONN16.46 245.11,130.81 245.11,142.24 246.38,143.51 CONN15.A29 246.38,149.86 245.11,151.13 245.11,163.83 246.38,165.1 CONN14.A29 246.38,170.18 245.11,171.45 245.11,184.15 246.38,185.42 CONN13.A29 246.38,190.5 245.11,191.77 245.11,204.47 246.38,205.74 CONN12.A29
!SCD0
  Bottom 0.305: CONN1.46 106.68,8.89 106.68,12.06 109.22,14.61 109.22,16.51 RES12.4 125.73,33.02 153.67,33.02 157.48,36.83 160.02,36.83 U41.32
!SCSI  (via drill 0.33)
  Top 0.305: v162.56,87 162.56,59.69 U40.8
  Route2 0.305: U38.3 167.64,109.22 162.56,109.22 | 162.56,109.22 162.56,114.3 160.02,116.84 160.02,118.75 160.66,119.38 162.56,119.38 U37.16 | 162.56,109.22 v162.56,87
!SCSI1  (via drill 0.33)
  Route2 0.305: U57.24 271.78,77.47 v271.78,64.77 | v175.26,63.5 172.72,63.5 170.18,60.96 170.18,57.15 166.37,53.34 161.29,53.34 U40.12
  Bottom 0.305: v271.78,64.77 237.49,64.77 236.22,66.04 215.9,66.04 214.63,64.77 185.42,64.77 184.15,63.5 v175.26,63.5
!SCSII0  (via drill 0.33)
  Route2 0.305: v232.41,55.88 234.95,55.88 236.22,57.15 U46.35
  Route15 0.305: RES13.8 147.32,69.85 147.32,62.87 150.5,59.69 174.62,59.69 175.26,59.05 175.26,57.15 176.53,55.88 | 176.53,55.88 U40.1 182.88,54.61 222.25,54.61 223.52,55.88 v232.41,55.88 | 176.53,55.88 172.72,52.07 172.72,38.73 176.53,34.92 U41.57
!SD00
  Route2 0.305: U41.38 162.56,29.21 162.56,8.89 CONN1.2
  Bottom 0.305: U41.38 160.02,29.21 149.86,29.21 RES14.5
!SD0
  Top 0.305: U57.10 289.56,90.17 289.56,92.71 292.1,95.25 292.1,105.41 RES18.1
